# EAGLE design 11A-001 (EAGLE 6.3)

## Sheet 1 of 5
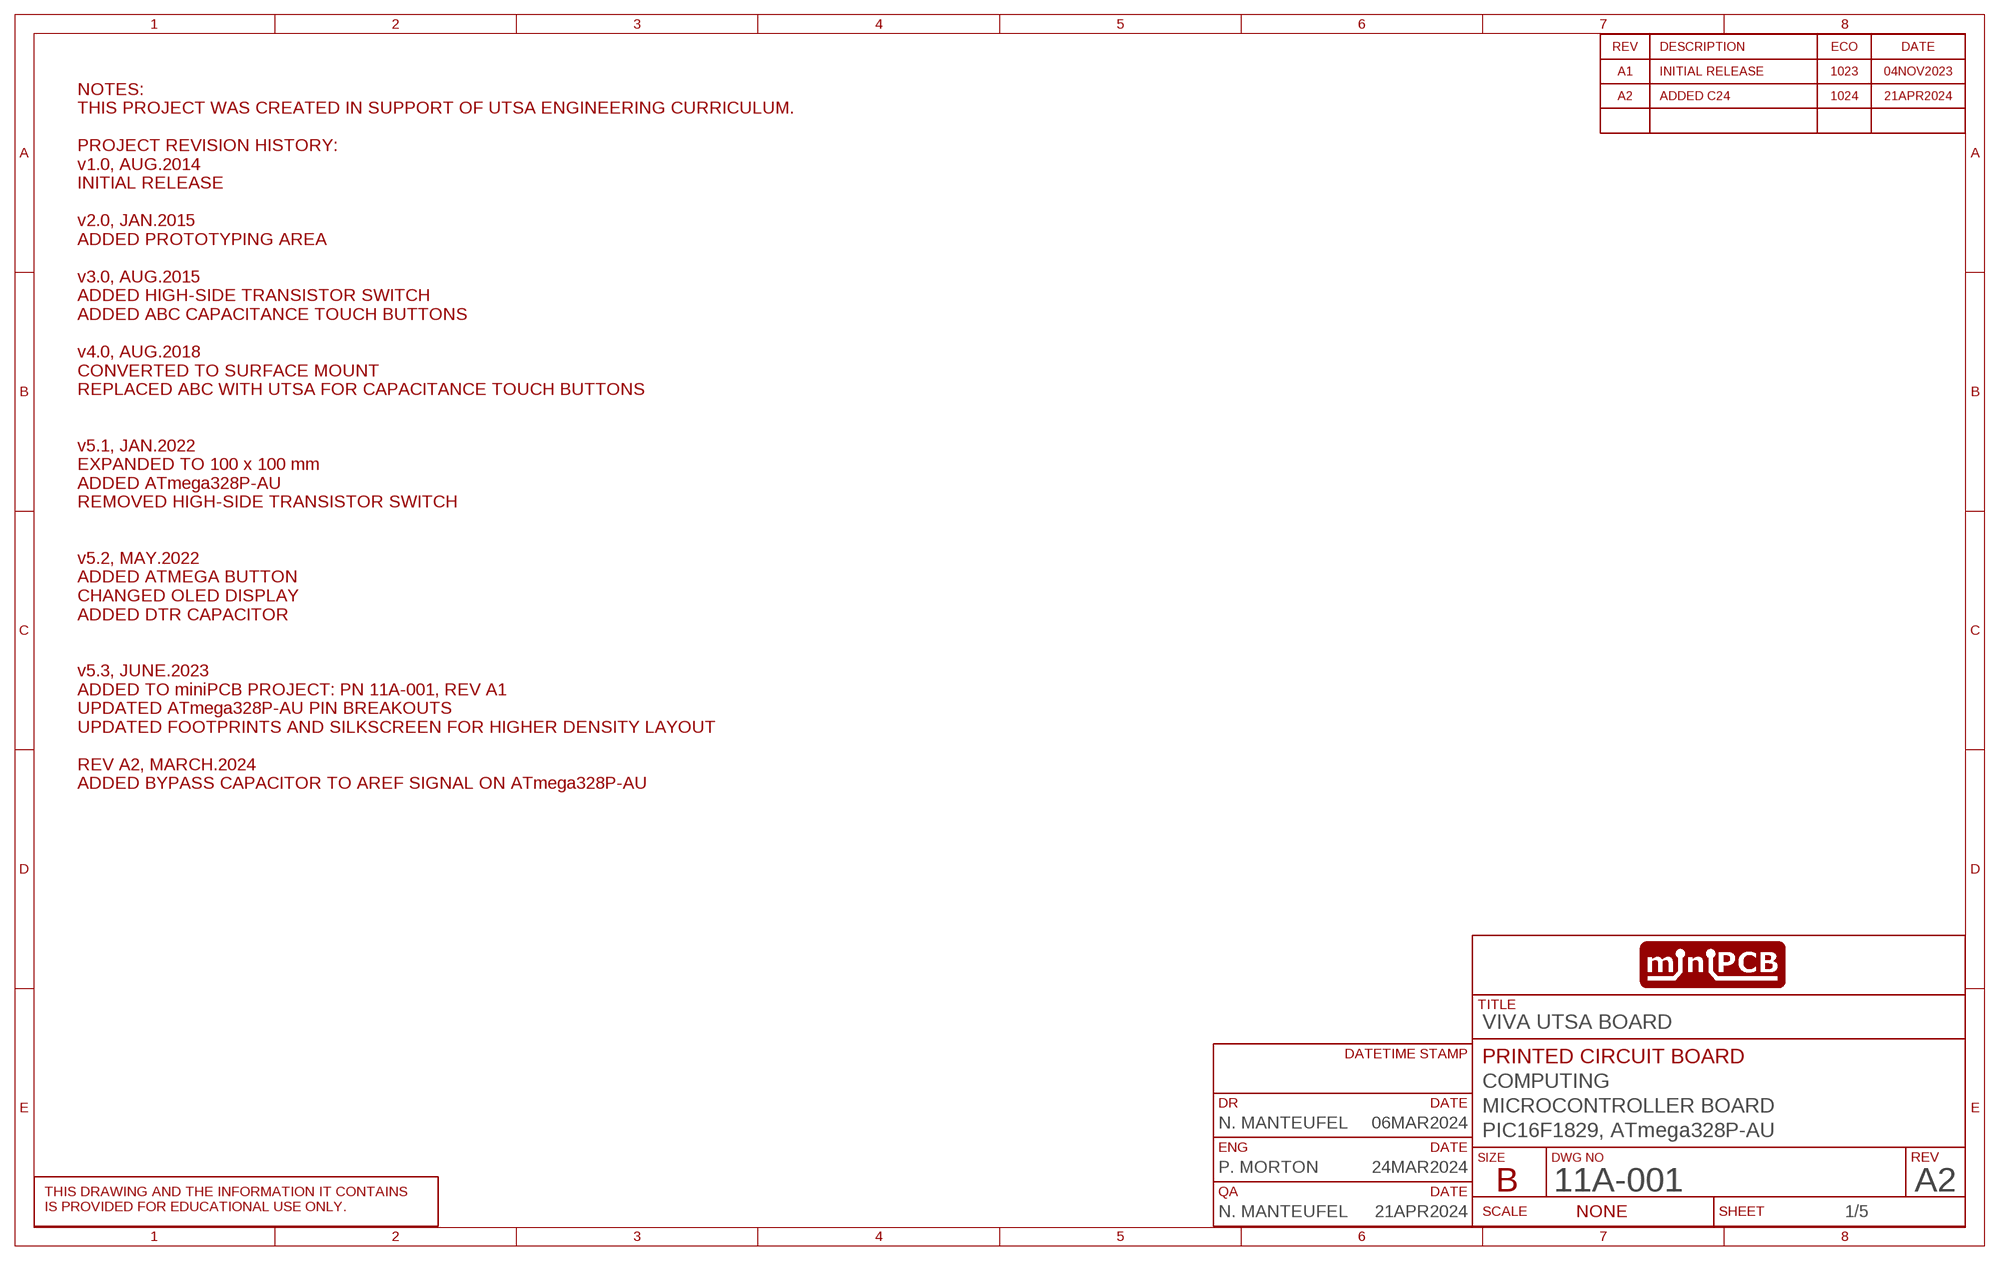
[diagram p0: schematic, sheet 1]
SHEET1 (SCHEMATIC): CIRCUIT_CATEGORY: COMPUTING; CIRCUIT_NAME: MICROCONTROLLER BOARD; CIRCUIT_VARIANT: PIC16F1829, ATmega328P-AU; DR: N. MANTEUFEL; DR_DATE: 06MAR2024; ENG: P. MORTON; ENG_DATE: 24MAR2024; PCB_PCBA: PRINTED CIRCUIT BOARD; QA: N. MANTEUFEL; QA_DATE: 21APR2024; REVA: A1; REVA_DATE: 04NOV2023; REVA_ECO: 1023; REVB: A2; REVB_DATE: 21APR2024; REVB_DESCRIPTION: ADDED C24; REVB_ECO: 1024; REVISION: A2; TITLE: VIVA UTSA BOARD

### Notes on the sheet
- NOTES:
  THIS PROJECT WAS CREATED IN SUPPORT OF UTSA ENGINEERING CURRICULUM.
  
  PROJECT REVISION HISTORY:
  v1.0, AUG.2014
  INITIAL RELEASE
  
  v2.0, JAN.2015
  ADDED PROTOTYPING AREA
  
  v3.0, AUG.2015
  ADDED HIGH-SIDE TRANSISTOR SWITCH
  ADDED ABC CAPACITANCE TOUCH BUTTONS
  
  v4.0, AUG.2018
  CONVERTED TO SURFACE MOUNT
  REPLACED ABC WITH UTSA FOR CAPACITANCE TOUCH BUTTONS
  
  
  v5.1, JAN.2022
  EXPANDED TO 100 x 100 mm
  ADDED ATmega328P-AU
  REMOVED HIGH-SIDE TRANSISTOR SWITCH
  
  
  v5.2, MAY.2022
  ADDED ATMEGA BUTTON
  CHANGED OLED DISPLAY
  ADDED DTR CAPACITOR
  
  
  v5.3, JUNE.2023
  ADDED TO miniPCB PROJECT: PN 11A-001, REV A1
  UPDATED ATmega328P-AU PIN BREAKOUTS
  UPDATED FOOTPRINTS AND SILKSCREEN FOR HIGHER DENSITY LAYOUT
  
  REV A2, MARCH.2024
  ADDED BYPASS CAPACITOR TO AREF SIGNAL ON ATmega328P-AU

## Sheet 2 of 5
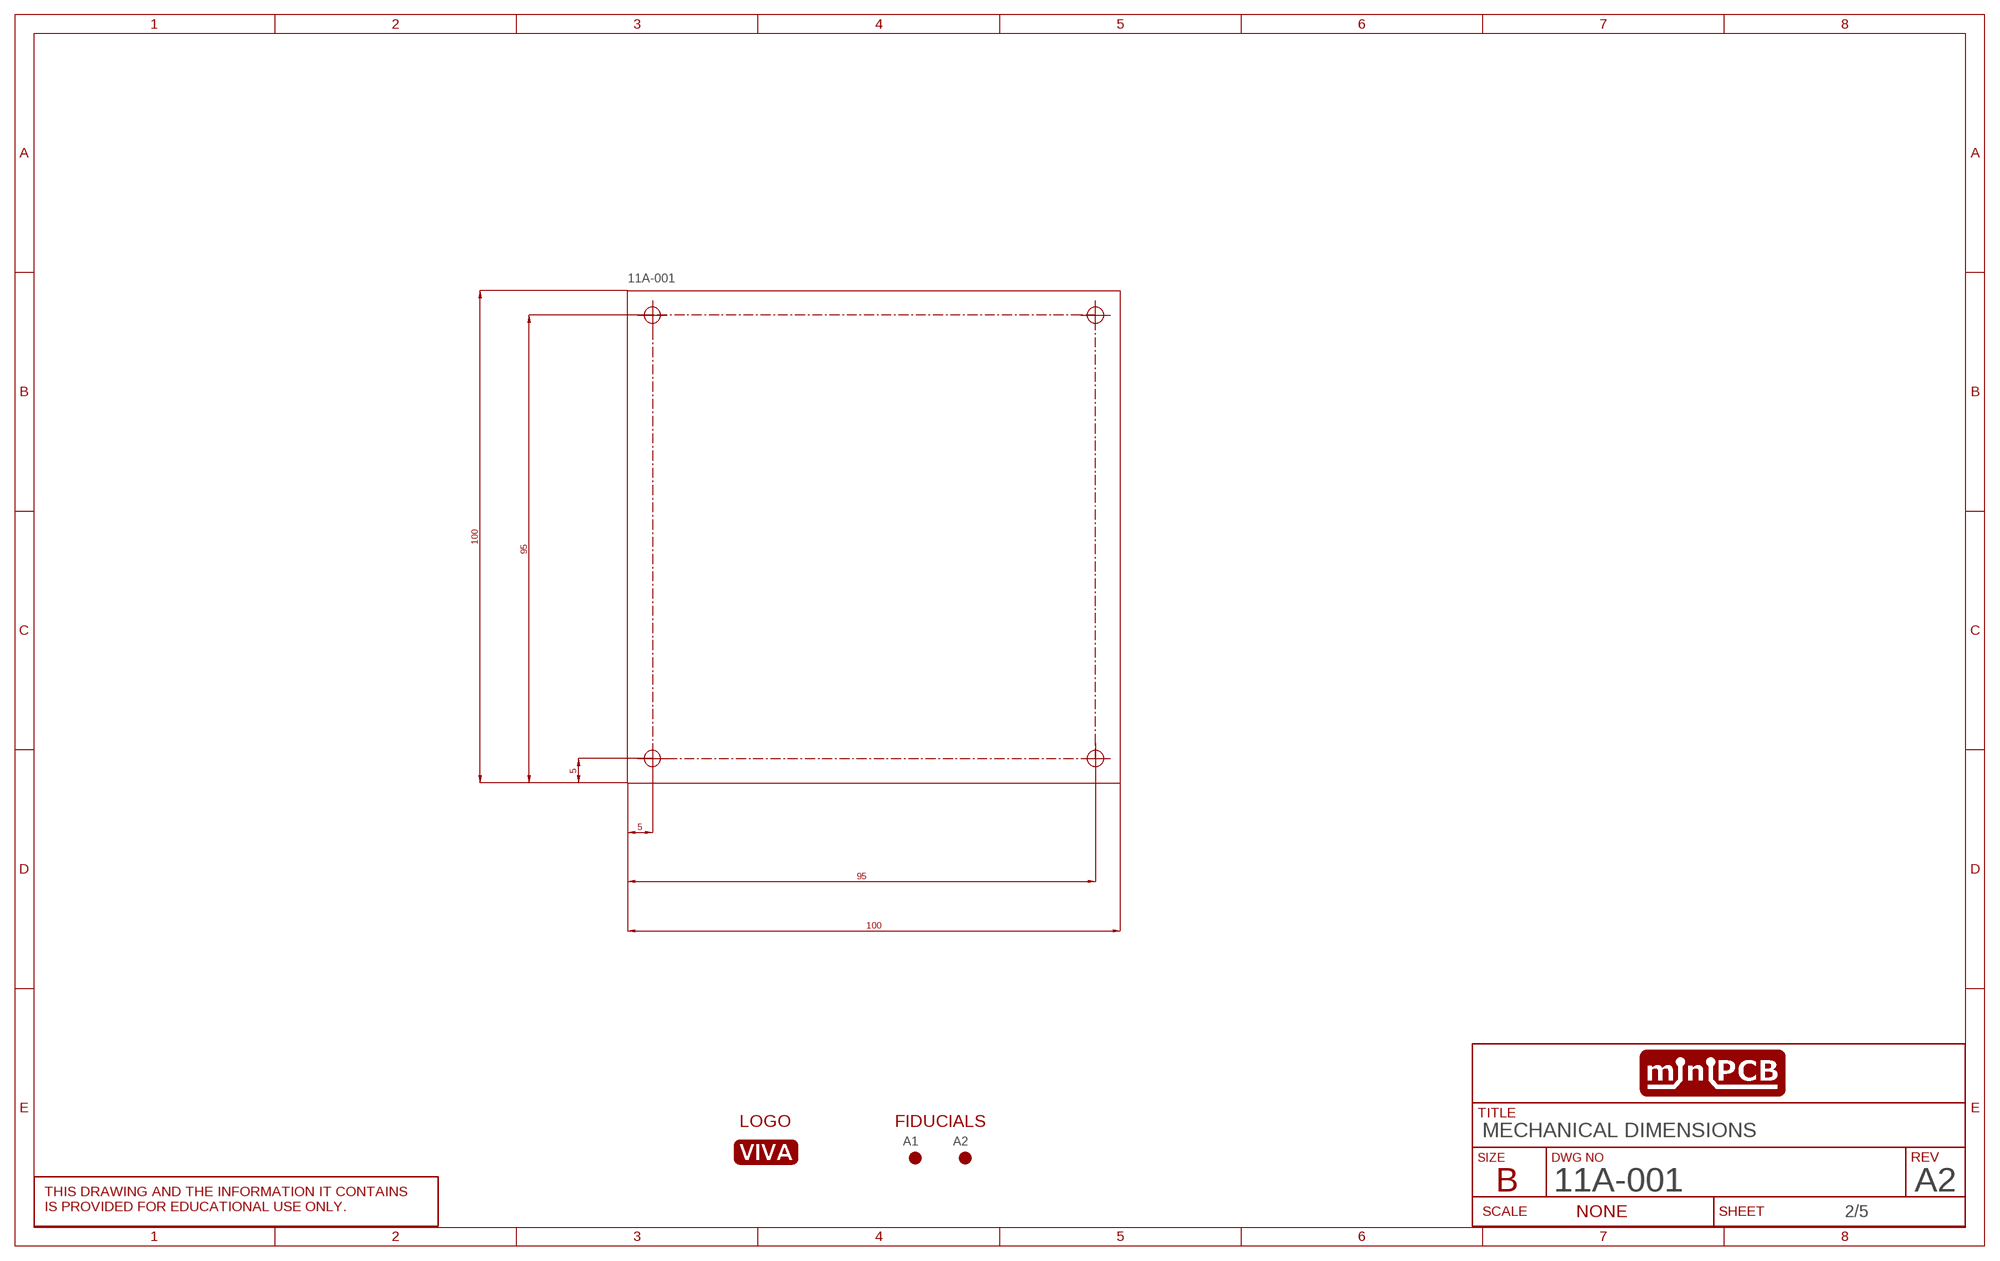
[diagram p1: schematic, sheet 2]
SHEET2 (SCHEMATIC): CIRCUIT_CATEGORY: COMPUTING; CIRCUIT_NAME: MICROCONTROLLER BOARD; CIRCUIT_VARIANT: PIC16F1829, ATmega328P-AU; DR: N. MANTEUFEL; DR_DATE: 31JUL2023; ENG: P. MORTON; ENG_DATE: 31JUL2023; PCB_PCBA: PRINTED CIRCUIT BOARD; REVA: A; REVISION: A2; TITLE: MECHANICAL DIMENSIONS

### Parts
-  11A-001  PCB_100X100  [PCB_100X100]
A1  FIDUCIAL  [FIDUCIAL]
A2  FIDUCIAL  [FIDUCIAL]
U$2  VIVA_LOGO  [VIVA_LOGO]

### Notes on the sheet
- LOGO | FIDUCIALS

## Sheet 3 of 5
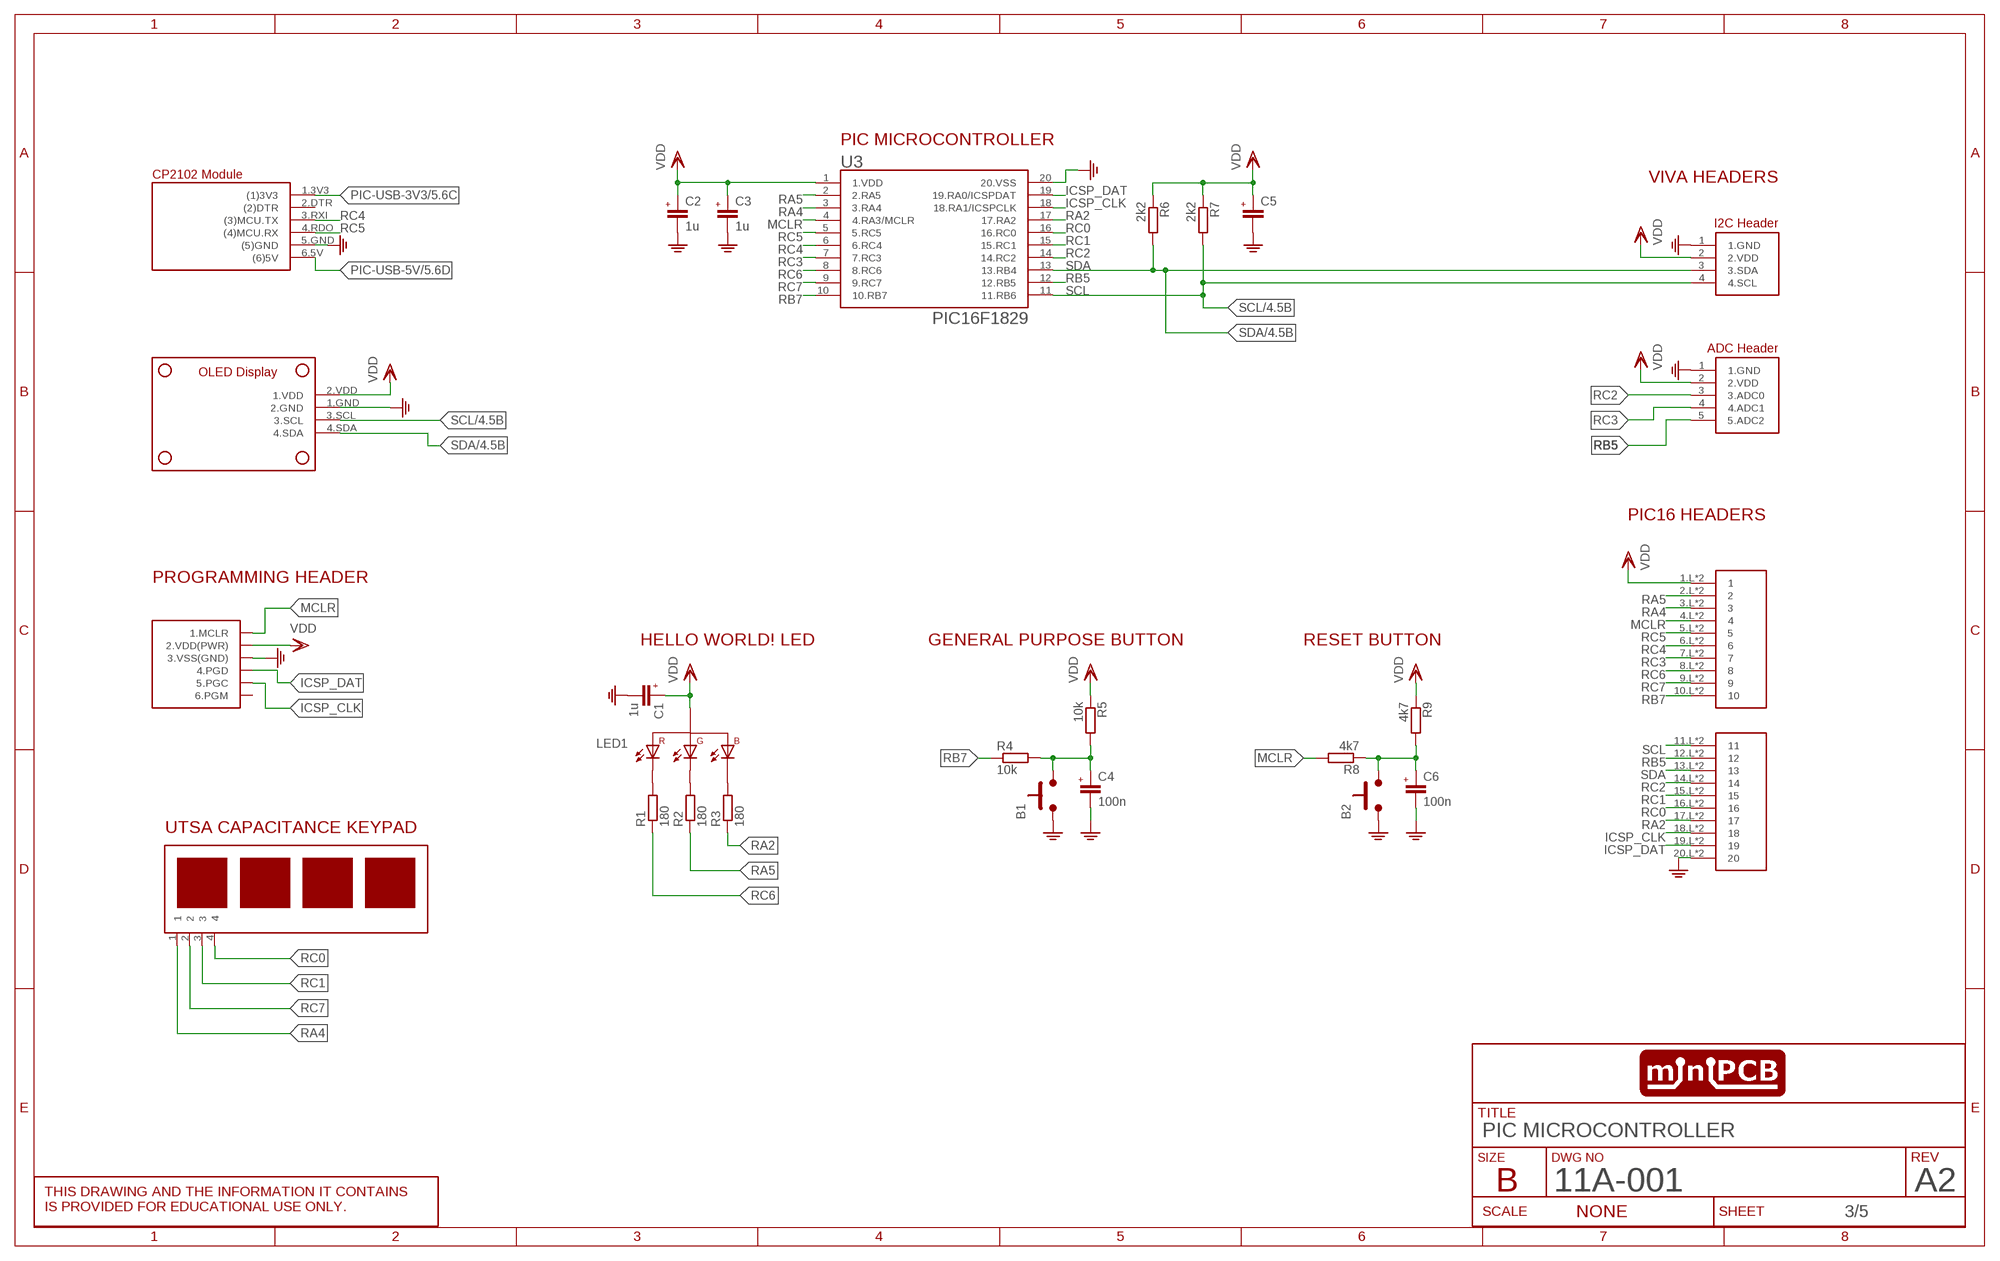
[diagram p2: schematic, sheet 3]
SHEET3 (SCHEMATIC): CIRCUIT_CATEGORY: COMPUTING; CIRCUIT_NAME: MICROCONTROLLER BOARD; CIRCUIT_VARIANT: PIC16F1829, ATmega328P-AU; DR: N. MANTEUFEL; DR_DATE: 31JUL2023; ENG: P. MORTON; ENG_DATE: 31JUL2023; PCB_PCBA: PRINTED CIRCUIT BOARD; REVA: A; REVISION: A2; TITLE: PIC MICROCONTROLLER

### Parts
$3_73_$  VIVA_OLEDGND  [VIVA_OLED-I2C-ALT]
B1  PUSHBUTTON6X6MM  [6X6MM]
B2  PUSHBUTTON6X6MM  [6X6MM]
C1  1u  C0805  [C0805]
C2  1u  C0805  [C0805]
C3  1u  C0805  [C0805]
C4  100n  C0805  [C0805]
C5  C0805  [C0805]
C6  100n  C0805  [C0805]
J1  PICKIT3  [PICKIT3]
J2  VIVA-HEADER-ADC-PIC16  [VIVA-HEADER-ADC-PIC16]
LED1  LED_RGBLTST-C19FD1WT  [0805_RGB]
R1  180  R-EU__R0805  [R0805]
R2  180  R-EU__R0805  [R0805]
R3  180  R-EU__R0805  [R0805]
R4  10k  R-EU__R0805  [R0805]
R5  10k  R-EU__R0805  [R0805]
R6  2k2  R-EU__R0805  [R0805]
R7  2k2  R-EU__R0805  [R0805]
R8  4k7  R-EU__R0805  [R0805]
R9  4k7  R-EU__R0805  [R0805]
U1  VIVA_UTSA-KEYPADV5  [VIVA_UTSA-KEYPAD-V5]
U2  VIVA_USB-TTL  [VIVA_USB_TTL_SUBTEXT]
U3  PIC16F1829  PIC16F1829300  [SOP20-NEW]
U4  VIVA-HEADER-I2C-RA  [VIVA-HEADER-I2C-RA]
U5  VIVA_PIC16BOARD  [VIVA_PIC16]

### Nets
B1-CAP: B1.3.B B1.4.B C4.1(+) R4.2 R5.2
GND: $3_73_$.1.GND(2.GND) B1.1.A B1.2.A B2.1.A B2.2.A C1.2(-) C2.2(-) C3.2(-) C4.2(-) C5.2(-) C6.2(-) J1.3(3.VSS(GND)) J2.1(1.GND) U2.5.GND((5)GND) U3.20(20.VSS) U4.1(1.GND) U5.20.L U5.20.R ; also sheet 4,5
ICSP_CLK: J1.5(5.PGC) U3.18(18.RA1/ICSPCLK) U5.18.L U5.18.R
ICSP_DAT: J1.4(4.PGD) U3.19(19.RA0/ICSPDAT) U5.19.L U5.19.R
MCLR: J1.1(1.MCLR) R8.2 U3.4(4.RA3/MCLR) U5.4.L U5.4.R
MCLR_CAP: B2.3.B B2.4.B C6.1(+) R8.1 R9.2
N$4: LED1.2(1.R-) R1.2
N$5: LED1.3(2.G-) R2.2
N$6: LED1.1(4.B-) R3.2
PIC-USB-3V3: U2.1.3V3((1)3V3) ; also sheet 5
PIC-USB-5V: U2.6.5V((6)5V) ; also sheet 5
RA2: R3.1 U3.17(17.RA2) U5.17.L U5.17.R
RA4: U1.1 U3.3(3.RA4) U5.3.L U5.3.R
RA5: R2.1 U3.2(2.RA5) U5.2.L U5.2.R
RB5: J2.5(5.ADC2) U3.12(12.RB5) U5.12.L U5.12.R
RB7: R4.1 U3.10(10.RB7) U5.10.L U5.10.R
RC0: U1.4 U3.16(16.RC0) U5.16.L U5.16.R
RC1: U1.3 U3.15(15.RC1) U5.15.L U5.15.R
RC2: J2.3(3.ADC0) U3.14(14.RC2) U5.14.L U5.14.R
RC3: J2.4(4.ADC1) U3.7(7.RC3) U5.7.L U5.7.R
RC4: U2.3.RXI((3)MCU.TX) U3.6(6.RC4) U5.6.L U5.6.R
RC5: U2.4.RDO((4)MCU.RX) U3.5(5.RC5) U5.5.L U5.5.R
RC6: R1.1 U3.8(8.RC6) U5.8.L U5.8.R
RC7: U1.2 U3.9(9.RC7) U5.9.L U5.9.R
SCL: $3_73_$.3.SCL R7.2 U3.11(11.RB6) U4.4(4.SCL) U5.11.L U5.11.R ; also sheet 4
SDA: $3_73_$.4.SDA R6.2 U3.13(13.RB4) U4.3(3.SDA) U5.13.L U5.13.R ; also sheet 4
VDD: $3_73_$.2.VDD(1.VDD) C1.1(+) C2.1(+) C3.1(+) C5.1(+) J1.2(2.VDD(PWR)) J2.2(2.VDD) LED1.4(3.+) R5.1 R6.1 R7.1 R9.1 U3.1(1.VDD) U4.2(2.VDD) U5.1.L U5.1.R ; also sheet 4,5
Unconnected: J1.6(6.PGM) U2.2.DTR((2)DTR)

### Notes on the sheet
- PIC MICROCONTROLLER
- VIVA HEADERS
- PIC16 HEADERS
- PROGRAMMING HEADER
- HELLO WORLD! LED | GENERAL PURPOSE BUTTON | RESET BUTTON
- UTSA CAPACITANCE KEYPAD

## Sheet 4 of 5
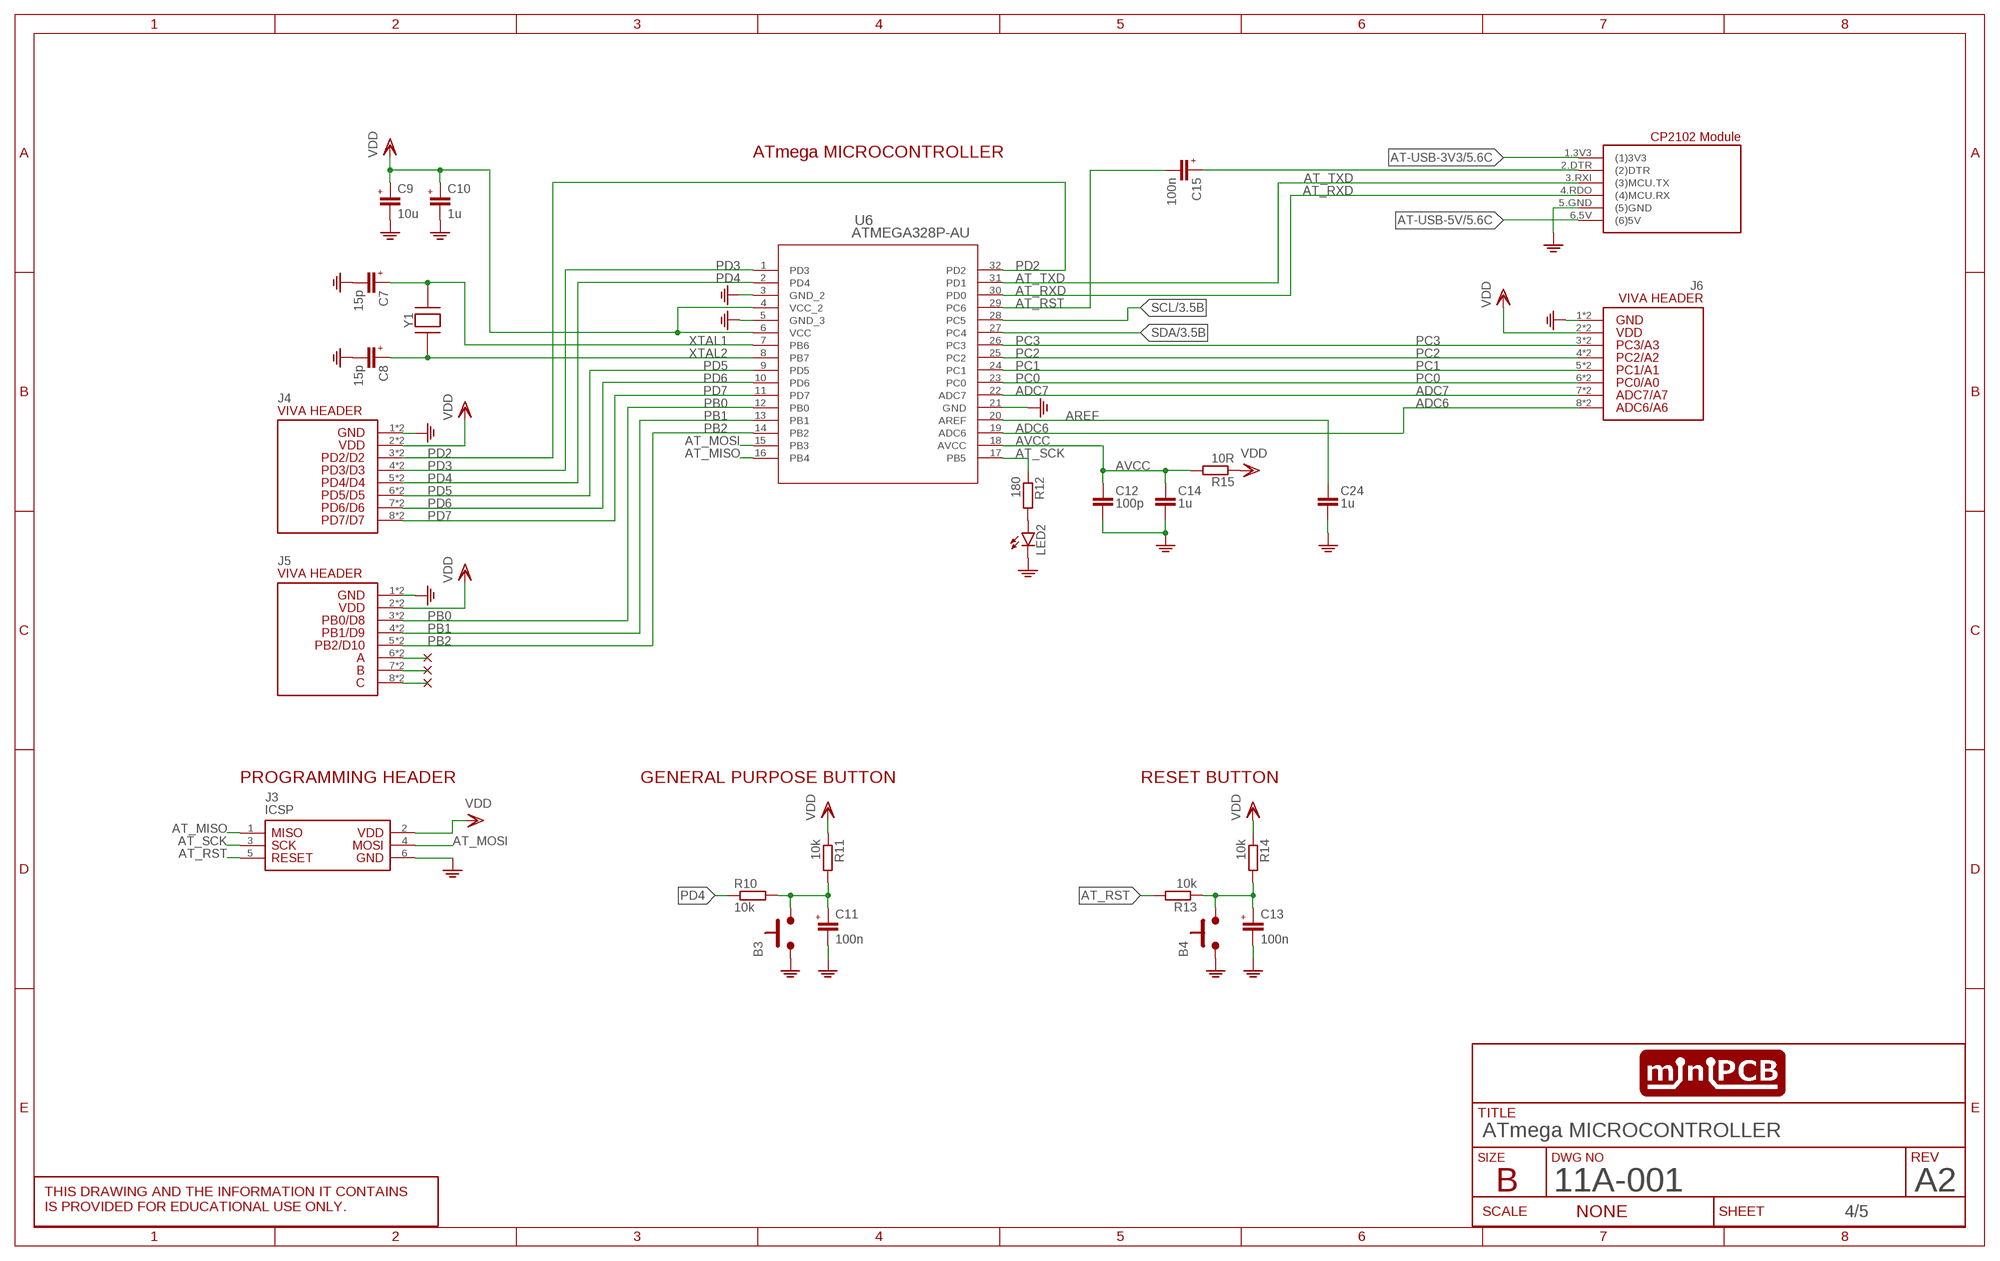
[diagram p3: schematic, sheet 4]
SHEET4 (SCHEMATIC): CIRCUIT_CATEGORY: COMPUTING; CIRCUIT_NAME: MICROCONTROLLER BOARD; CIRCUIT_VARIANT: PIC16F1829, ATmega328P-AU; DR: N. MANTEUFEL; DR_DATE: 31JUL2023; ENG: P. MORTON; ENG_DATE: 31JUL2023; PCB_PCBA: PRINTED CIRCUIT BOARD; REVA: A; REVISION: A2; TITLE: ATmega MICROCONTROLLER

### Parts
B3  PUSHBUTTON6X6MM  [6X6MM]
B4  PUSHBUTTON6X6MM  [6X6MM]
C7  15p  C0603  [C0603]
C8  15p  C0603  [C0603]
C9  10u  C0805  [C0805]
C10  1u  C0805  [C0805]
C11  100n  C0805  [C0805]
C12  100p  C-EU_C0805  [C0805]
C13  100n  C0805  [C0805]
C14  1u  C-EU_C0805  [C0805]
C15  100n  C0805  [C0805]
C24  1u  C-EU_C0805  [C0805]
J3  ICSP  PINS_6-2X3_AT  [PINS_6-2X3_AT]
J4  VIVA-HEADER-ADC-8P  [VIVA-HEADER-ADC-8P]
J5  VIVA-HEADER-ADC-8P  [VIVA-HEADER-ADC-8P]
J6  VIVA-HEADER-ADC-8P  [VIVA-HEADER-ADC-8P]
LED2  LEDSML0805  [SML0805]
R10  10k  R-EU__R0805  [R0805]
R11  10k  R-EU__R0805  [R0805]
R12  180  R-EU__R0805  [R0805]
R13  10k  R-EU__R0805  [R0805]
R14  10k  R-EU__R0805  [R0805]
R15  10R  R-EU__R0805  [R0805]
U6  ATMEGA328P-AU  ATMEGA328-AU  [32A_ATM]
U7  VIVA_USB-TTL  [VIVA_USB_TTL_SUBTEXT]
Y1  CRYSTAL-3225_4P  [TXC7M2]

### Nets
ADC6: J6.8(8.ADC5) J6.9(8.ADC5) U6.19(ADC6)
ADC7: J6.7(7.ADC4) J6.10(7.ADC4) U6.22(ADC7)
AREF: C24.1 U6.20(AREF)
AT-USB-3V3: U7.1.3V3((1)3V3) ; also sheet 5
AT-USB-5V: U7.6.5V((6)5V) ; also sheet 5
AT_DTR_CAP: C15.1(+) U7.2.DTR((2)DTR)
AT_MISO: J3.1 U6.16(PB4)
AT_MOSI: J3.4 U6.15(PB3)
AT_RST: C15.2(-) J3.5 R13.2 U6.29(PC6)
AT_RST_CAP: B4.3.B B4.4.B C13.1(+) R13.1 R14.2
AT_RXD: U6.30(PD0) U7.4.RDO((4)MCU.RX)
AT_SCK: J3.3 R12.1 U6.17(PB5)
AT_TXD: U6.31(PD1) U7.3.RXI((3)MCU.TX)
AVCC: C12.1 C14.1 R15.2 U6.18(AVCC)
GND: B3.1.A B3.2.A B4.1.A B4.2.A C7.1(-) C8.1(-) C9.2(-) C10.2(-) C11.2(-) C12.2 C13.2(-) C14.2 C24.2 J3.6 J4.1(1.GND) J4.16(1.GND) J5.1(1.GND) J5.16(1.GND) J6.1(1.GND) J6.16(1.GND) LED2.C U6.3(GND_2) U6.5(GND_3) U6.21(GND) U7.5.GND((5)GND) ; also sheet 3,5
N$33: J5.6(6.ADC3) J5.11(6.ADC3)
N$34: J5.7(7.ADC4) J5.10(7.ADC4)
N$35: J5.8(8.ADC5) J5.9(8.ADC5)
N$37: LED2.A R12.2
PB0: J5.3(3.ADC0) J5.14(3.ADC0) U6.12(PB0)
PB1: J5.4(4.ADC1) J5.13(4.ADC1) U6.13(PB1)
PB2: J5.5(5.ADC2) J5.12(5.ADC2) U6.14(PB2)
PC0: J6.6(6.ADC3) J6.11(6.ADC3) U6.23(PC0)
PC1: J6.5(5.ADC2) J6.12(5.ADC2) U6.24(PC1)
PC2: J6.4(4.ADC1) J6.13(4.ADC1) U6.25(PC2)
PC3: J6.3(3.ADC0) J6.14(3.ADC0) U6.26(PC3)
PD2: J4.3(3.ADC0) J4.14(3.ADC0) U6.32(PD2)
PD3: J4.4(4.ADC1) J4.13(4.ADC1) U6.1(PD3)
PD4: J4.5(5.ADC2) J4.12(5.ADC2) R10.1 U6.2(PD4)
PD4-CAP: B3.3.B B3.4.B C11.1(+) R10.2 R11.2
PD5: J4.6(6.ADC3) J4.11(6.ADC3) U6.9(PD5)
PD6: J4.7(7.ADC4) J4.10(7.ADC4) U6.10(PD6)
PD7: J4.8(8.ADC5) J4.9(8.ADC5) U6.11(PD7)
SCL: U6.28(PC5) ; also sheet 3
SDA: U6.27(PC4) ; also sheet 3
VDD: C9.1(+) C10.1(+) J3.2 J4.2(2.VDD) J4.15(2.VDD) J5.2(2.VDD) J5.15(2.VDD) J6.2(2.VDD) J6.15(2.VDD) R11.1 R14.1 R15.1 U6.4(VCC_2) U6.6(VCC) ; also sheet 3,5
XTAL1: C7.2(+) U6.7(PB6) Y1.3
XTAL2: C8.2(+) U6.8(PB7) Y1.1

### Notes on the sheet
- ATmega MICROCONTROLLER
- PROGRAMMING HEADER | GENERAL PURPOSE BUTTON | RESET BUTTON

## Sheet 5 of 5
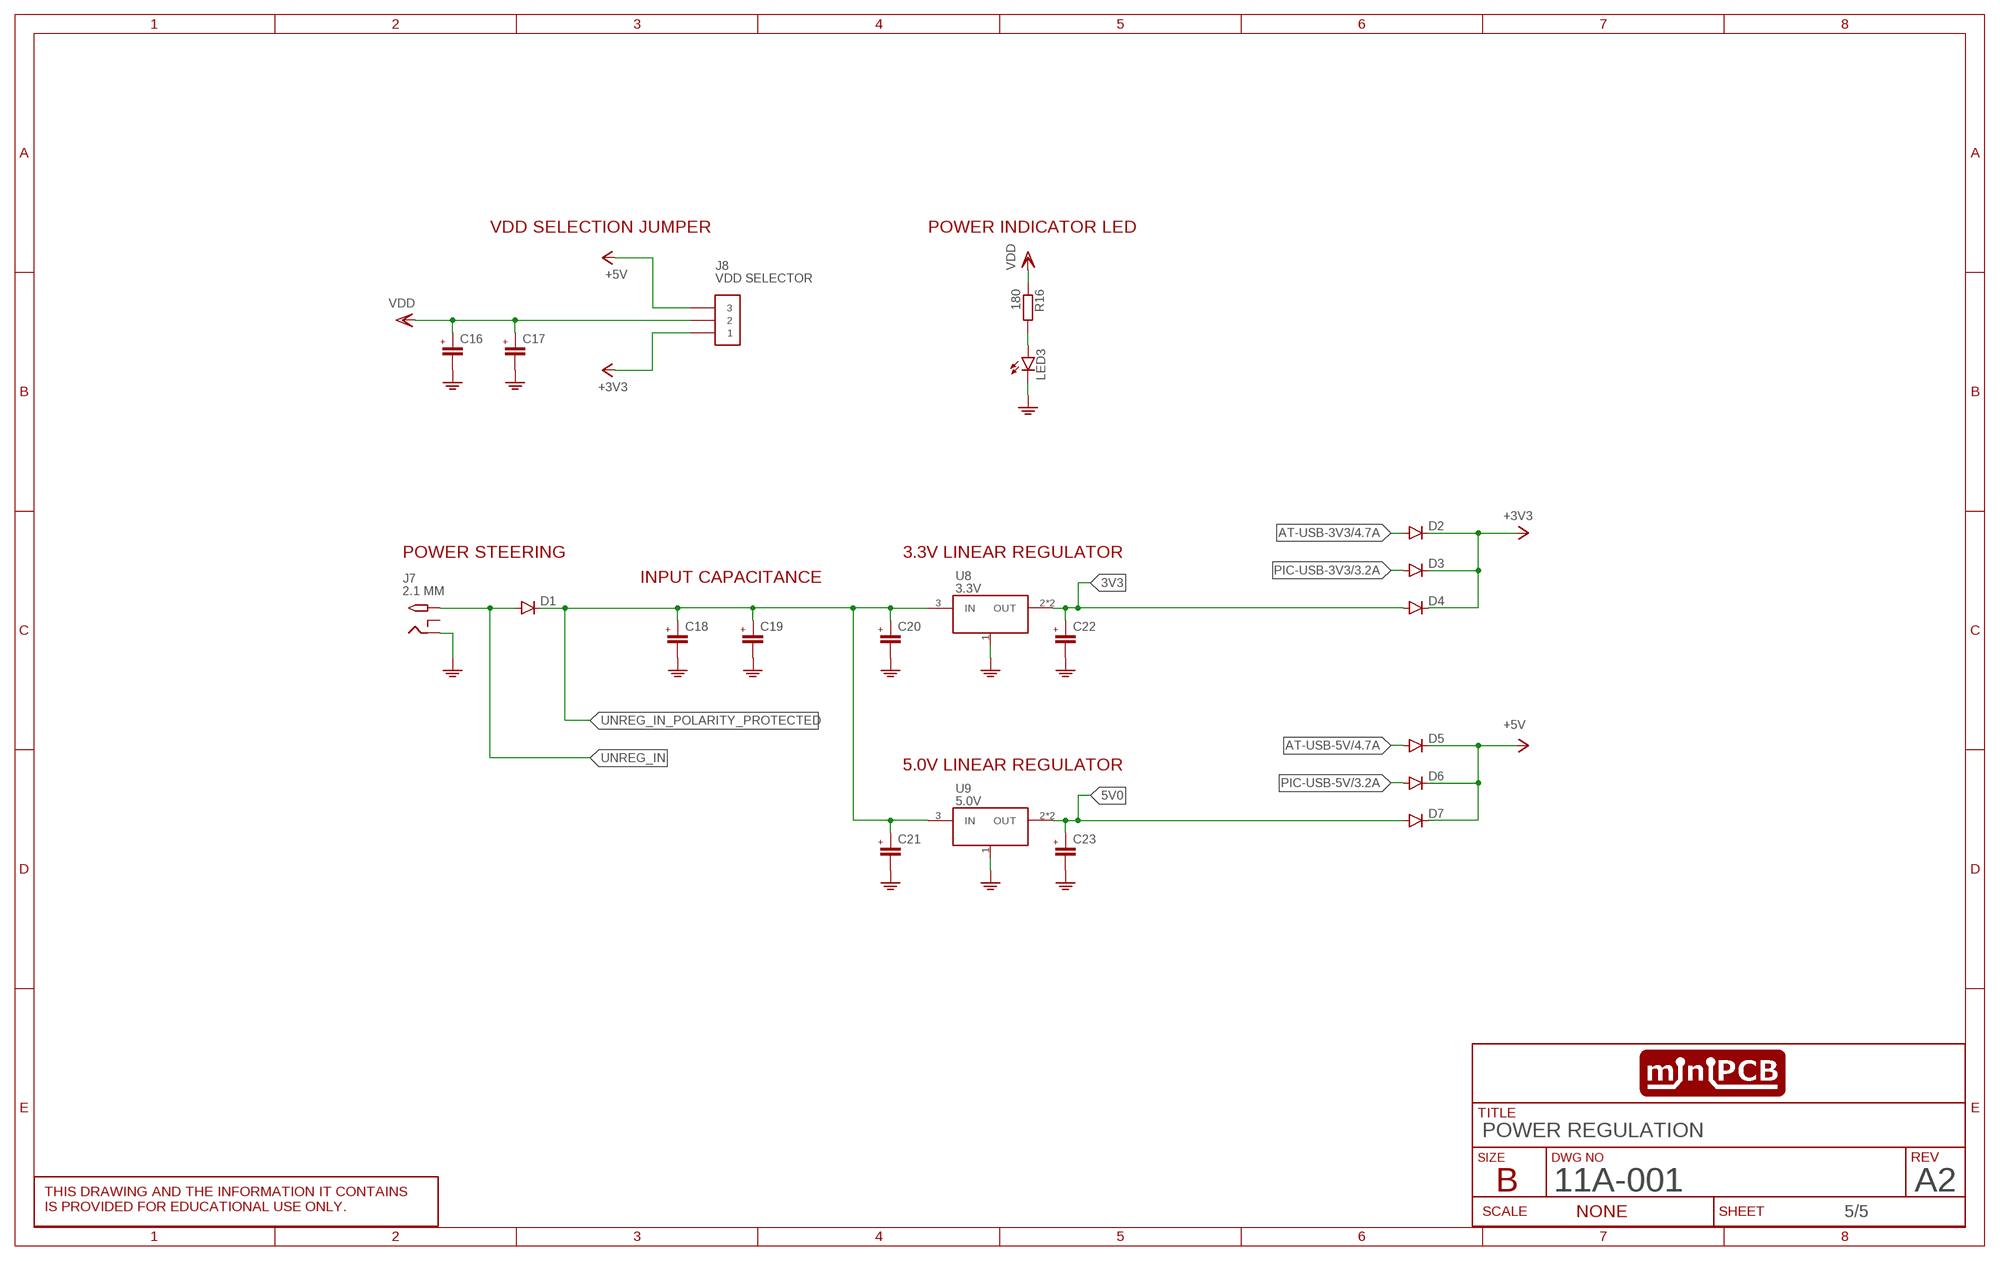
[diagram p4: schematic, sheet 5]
SHEET5 (SCHEMATIC): CIRCUIT_CATEGORY: COMPUTING; CIRCUIT_NAME: MICROCONTROLLER BOARD; CIRCUIT_VARIANT: PIC16F1829, ATmega328P-AU; DR: N. MANTEUFEL; DR_DATE: 31JUL2023; ENG: P. MORTON; ENG_DATE: 31JUL2023; PCB_PCBA: PRINTED CIRCUIT BOARD; REVA: A; REVISION: A2; TITLE: POWER REGULATION

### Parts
C16  C0805  [C0805]
C17  C0805  [C0805]
C18  C0805  [C0805]
C19  C0805  [C0805]
C20  C0805  [C0805]
C21  C0805  [C0805]
C22  C0805  [C0805]
C23  C0805  [C0805]
D1  DIODE-DO214AC  [DO214AC]
D2  DIODE-DO214AC  [DO214AC]
D3  DIODE-DO214AC  [DO214AC]
D4  DIODE-DO214AC  [DO214AC]
D5  DIODE-DO214AC  [DO214AC]
D6  DIODE-DO214AC  [DO214AC]
D7  DIODE-DO214AC  [DO214AC]
J7  2.1 MM  2.1MMJACKTHM  [PJ-102A]
J8  VDD SELECTOR  PINS_3_2.54  [PINS_3]
LED3  LEDSML0805  [SML0805]
R16  180  R-EU__R0805  [R0805]
U8  3.3V  REGULATOR_SCHLM1117  [SOT223]
U9  5.0V  REGULATOR_SCHLM1117  [SOT223]

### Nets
3V3: C22.1(+) D4.A U8.2(OUT) U8.4.TAB(OUT)
5V0: C23.1(+) D7.A U9.2(OUT) U9.4.TAB(OUT)
+3V3: D2.C D3.C D4.C J8.1
+5V: D5.C D6.C D7.C J8.3
AT-USB-3V3: D2.A ; also sheet 4
AT-USB-5V: D5.A ; also sheet 4
GND: C16.2(-) C17.2(-) C18.2(-) C19.2(-) C20.2(-) C21.2(-) C22.2(-) C23.2(-) J7.RING LED3.C U8.1(GND) U9.1(GND) ; also sheet 3,4
LED_POWER: LED3.A R16.2
PIC-USB-3V3: D3.A ; also sheet 3
PIC-USB-5V: D6.A ; also sheet 3
UNREG_IN: D1.A J7.TIP
UNREG_IN_POLARITY_PROTECTED: C18.1(+) C19.1(+) C20.1(+) C21.1(+) D1.C U8.3(IN) U9.3(IN)
VDD: C16.1(+) C17.1(+) J8.2 R16.1 ; also sheet 3,4
Unconnected: J7.RING_SW

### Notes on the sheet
- VDD SELECTION JUMPER | POWER INDICATOR LED
- POWER STEERING | 3.3V LINEAR REGULATOR
- INPUT CAPACITANCE
- 5.0V LINEAR REGULATOR

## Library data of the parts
$3_73_$ = utsa:VIVA_OLED
- = utsa:PCB_100X100
A1 A2 = utsa:FIDUCIAL
B1-B4 = nolan-utsa:PUSHBUTTON: Tactile push button switch
C1-C11 C13 C15-C23 = utsa:C
C12 C14 C24 = utsa:C-EU: CAPACITOR, European symbol
D1-D7 = utsa:DIODE-: DIODE
J1 = nolan-viva:PICKIT3
J2 = utsa:VIVA-HEADER-ADC
J3 = utsa:PINS_6-2X3_AT; P1: MISO; P2: VDD; P3: SCK; P4: MOSI; P5: RESET; P6: GND
J4 = utsa:VIVA-HEADER-ADC-8P; P3: PD2/D2; P4: PD3/D3; P5: PD4/D4; P6: PD5/D5; P7: PD6/D6; P8: PD7/D7
J5 = utsa:VIVA-HEADER-ADC-8P; P3: PB0/D8; P4: PB1/D9; P5: PB2/D10; P6: A; P7: B; P8: C
J6 = utsa:VIVA-HEADER-ADC-8P; P3: PC3/A3; P4: PC2/A2; P5: PC1/A1; P6: PC0/A0; P7: ADC7/A7; P8: ADC6/A6
J7 = utsa:2.1MMJACK: 2.1mm x 5.5mm THM DC jack with internal switch. Digikey part #PJ-102A, 4UCON part #05537 2.1mm x 5.5mm SMT DC jack with internal switch. Digikey part #PJ-002A-SMT, 4UCON part #03267 By microbuilder.eu & adafruit.com
J8 = utsa:PINS_3
LED1 = utsa:LED_RGB
LED2 LED3 = utsa:LED: LED
R1-R16 = utsa:R-EU_: RESISTOR, European symbol
U1 = utsa:VIVA_UTSA-KEYPAD
U2 U7 = utsa:VIVA_USB-TTL
U3 = utsa:PIC16F1829
U4 = utsa:VIVA-HEADER-I2C
U5 = utsa:VIVA_PIC16
U6 = utsa:ATMEGA328-AU; COPYRIGHT: Copyright (C) 2021 Ultra Librarian. All rights reserved.; MANUFACTURER_PART_NUMBER: ATMEGA328-AU; MFR_NAME: Microchip
U8 U9 = utsa:REGULATOR_SCH: Linear Regulator in SOT-223 package. NOTE: select correct pinout for your application. Tab may be OUT or GND!
U$2 = utsa:VIVA_LOGO
Y1 = utsa:CRYSTAL: HC49S Crystal Oscillator

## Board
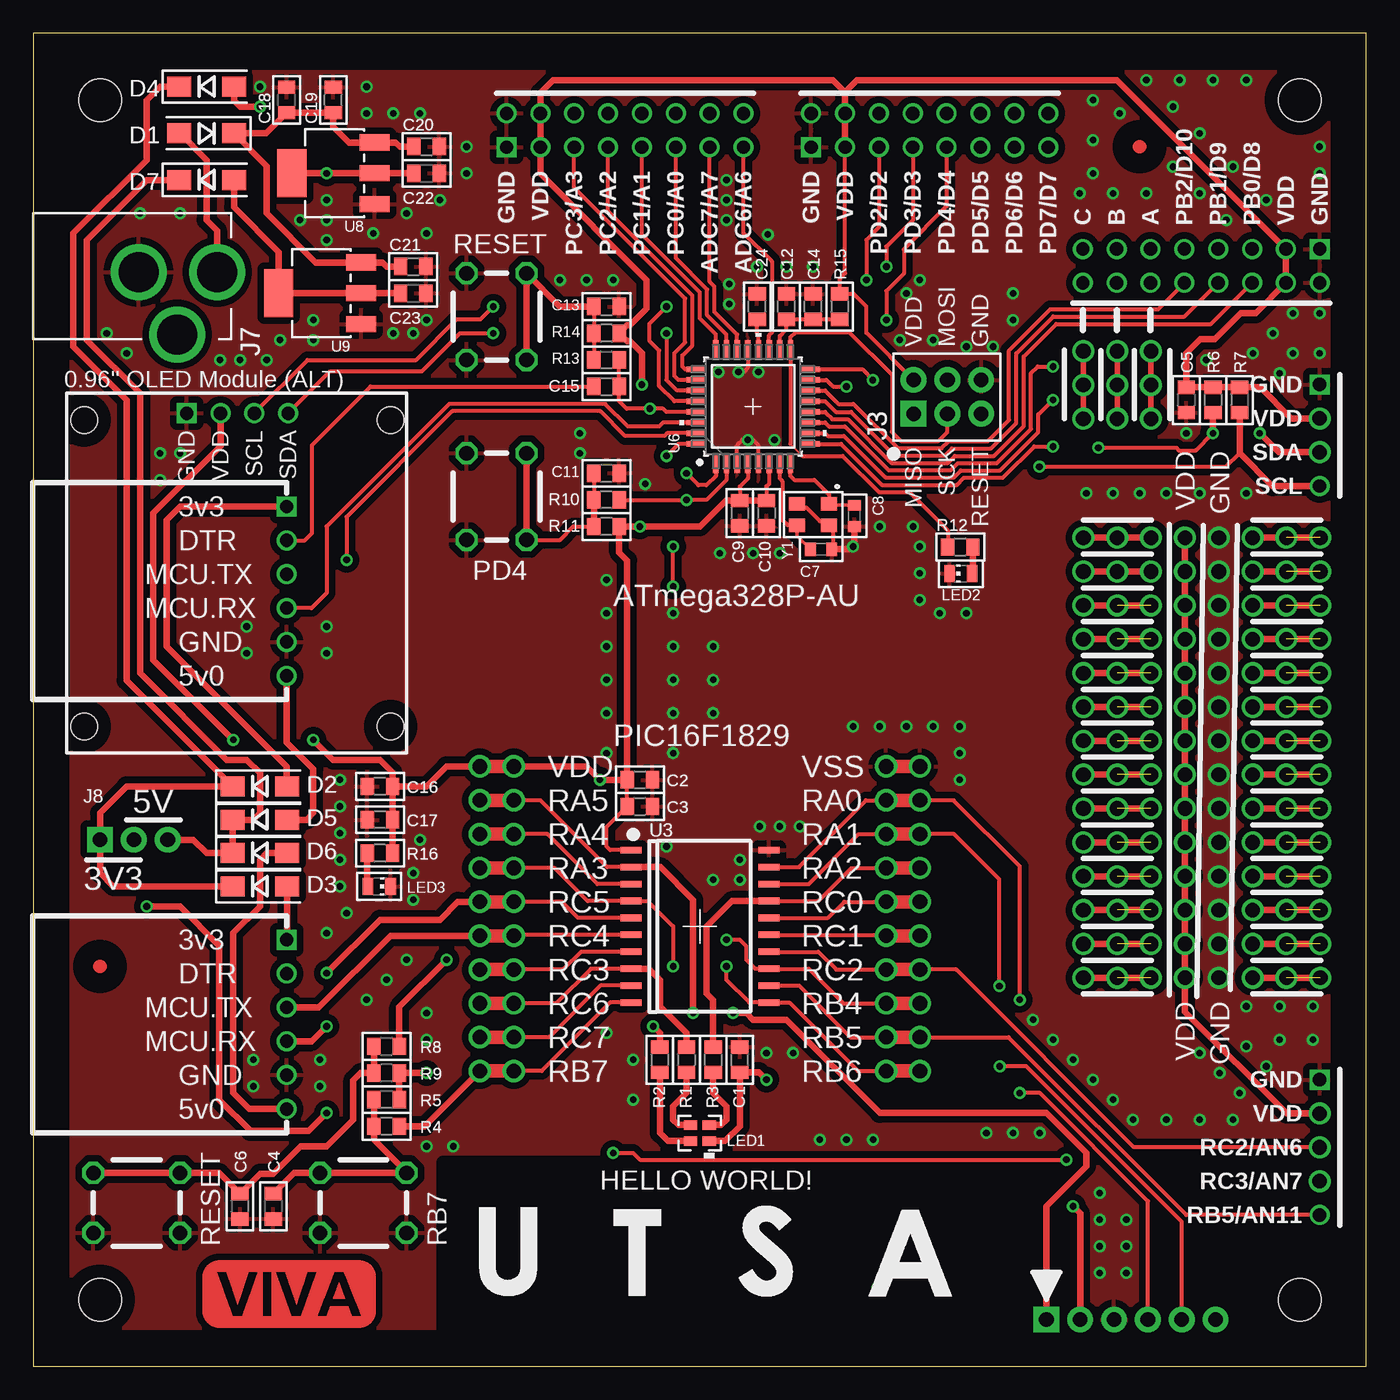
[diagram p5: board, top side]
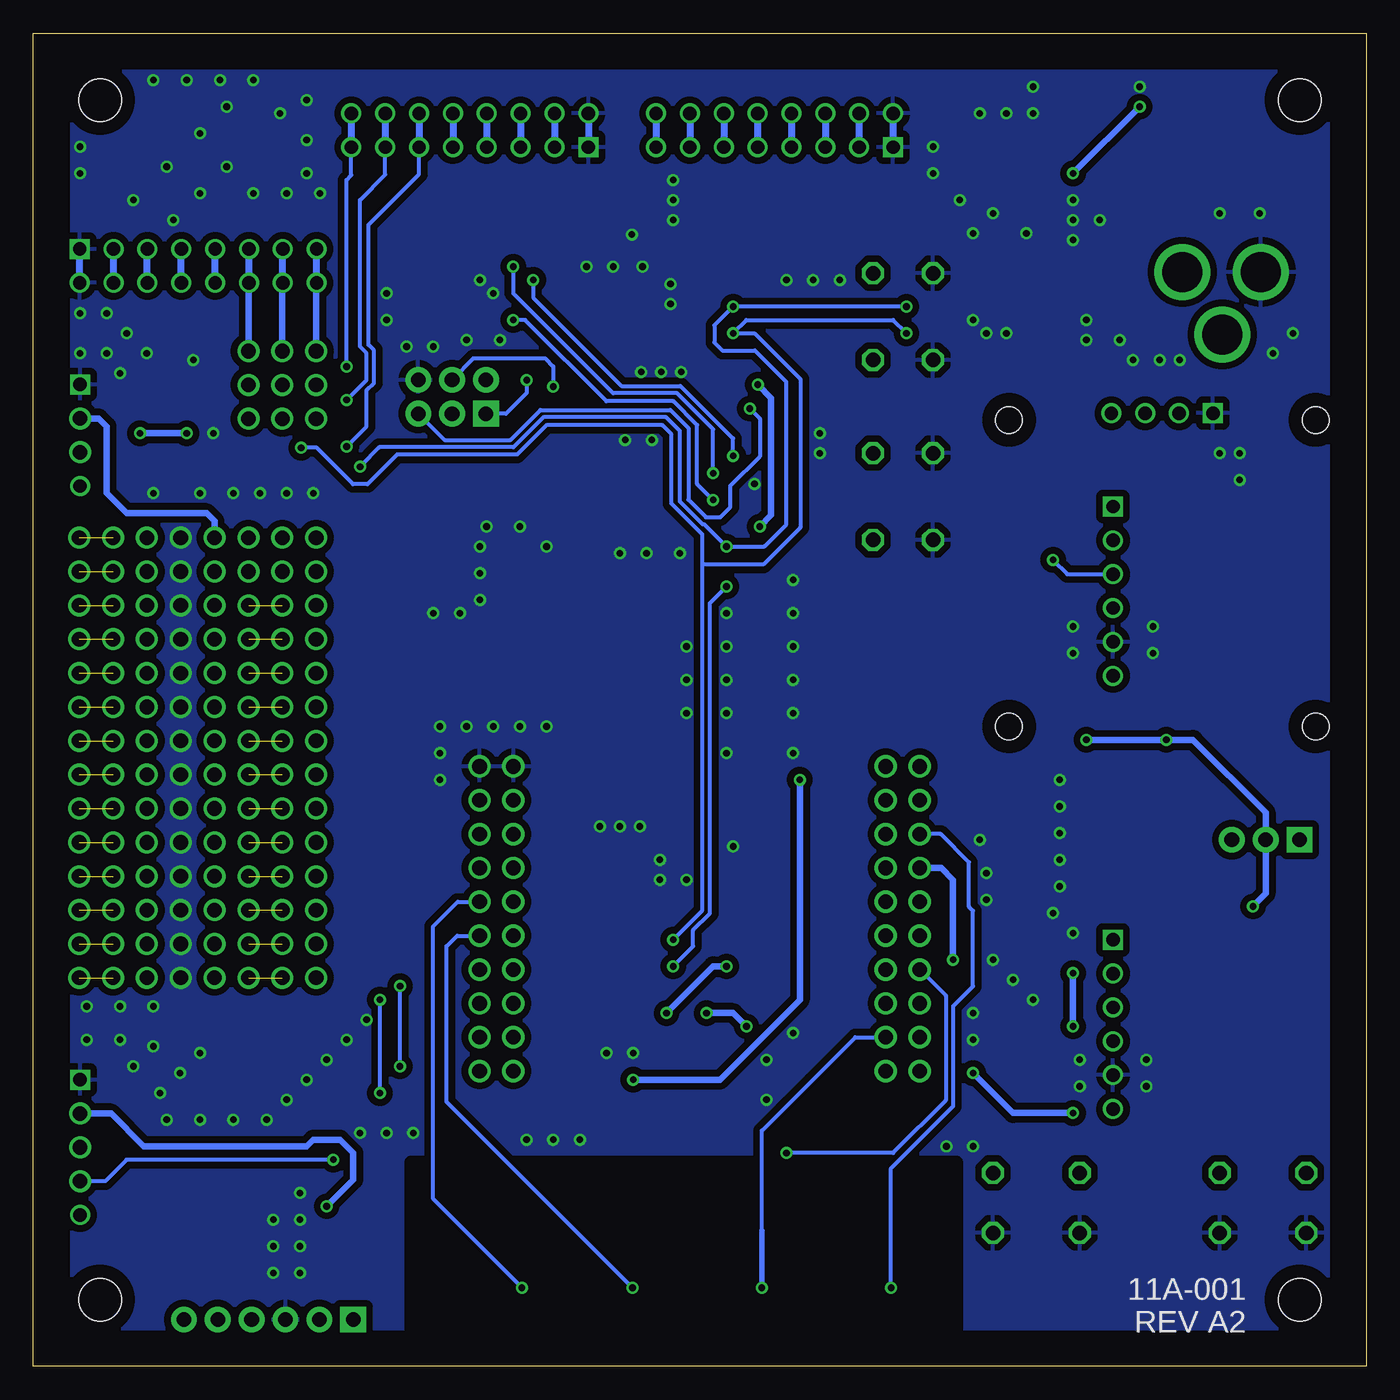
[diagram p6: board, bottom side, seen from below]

Size 100 x 100 mm. Coordinates in mm from the lower left corner, seen from the top.
Copper layers (1*16): Top 0.035mm / dielectric 1.5mm / Bottom 0.035mm
Design rules "minipcb": minimum track width 0.2mm, minimum drill 0.5mm, track to track 0.25mm, track to pad 0.5mm, pad to pad 0.5mm, via to via 0.5mm, smd to smd 0.15mm, copper to edge 1mm, drill to drill 1mm, minimum pad ring 0.2mm, minimum via ring 0.2mm, stop-mask expansion 0.1mm, vias tented up to drill 0.6mm, thermal gap 0.5mm

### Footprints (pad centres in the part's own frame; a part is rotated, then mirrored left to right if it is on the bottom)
VIVA_OLED-I2C-ALT = drill 1 square: 1.GND 0,0 | drill 1: 2.VDD 2.54,0; 3.SCL 5.08,0; 4.SDA 7.62,0 | hole 2: -7.7,-0.5; 15.3,-0.5; -7.7,-23.5; 15.3,-23.5
PCB_100X100 = hole 3.2: 5,95; 95,95; 95,5; 5,5
FIDUCIAL = smd 0 x 0: FIDUCIAL 0,0
6X6MM = drill 1.1 octagon: 1.A 0,0; 2.A 6.5,0; 3.B 0,4.5; 4.B 6.5,4.5
C0805 = smd 1 x 1.3: 1 -0.95,0; 2 0.95,0
C0603 = smd 0.8 x 1: 1 -0.8,0; 2 0.8,0
DO214AC = smd 1.8 x 1.5: A 2.05,0; C -2.05,0
PICKIT3 = drill 1.1 pad 1.93 square: 1 0,0 | drill 1.1 pad 1.93: 2 2.54,0; 3 5.08,0; 4 7.62,0; 5 10.16,0; 6 12.7,0
VIVA-HEADER-ADC-PIC16 = drill 1 square: 1 0,0 | drill 1.1: 2 2.54,0; 3 5.08,0; 4 7.62,0 | drill 1: 5 10.16,0
PINS_6-2X3_AT = drill 1.1 pad 1.93 square: 1 0,0 | drill 1.1 pad 1.93: 2 2.54,0; 3 0,-2.54; 4 2.54,-2.54; 5 0,-5.08; 6 2.54,-5.08
VIVA-HEADER-ADC-8P = drill 1 square: 1 0,0 | drill 1: 2 2.54,0; 3 5.08,0; 4 7.62,0; 5 10.16,0; 6 12.7,0; 7 15.24,0; 8 17.78,0; 9 17.78,2.54; 10 15.24,2.54; 11 12.7,2.54; 12 10.16,2.54; 13 7.62,2.54; 14 5.08,2.54; 15 2.54,2.54; 16 0,2.54
PJ-102A = drill 3 pad 4: RING 0.1,-3.39; RING_SW -4.6,-6.29; TIP 0.1,-9.29
PINS_3 = drill 1.1 pad 1.93 square: 1 0,0 | drill 1.1 pad 1.93: 2 2.54,0; 3 5.08,0
0805_RGB = smd 1 x 0.7: 1 0.7,0.6; 2 -0.7,0.6; 3 -0.7,-0.6; 4 0.7,-0.6
SML0805 = smd 0.8 x 1.27: A -0.9,0; C 0.8,0
R0805 = smd 1 x 1.3: 1 -0.95,0; 2 0.95,0
VIVA_UTSA-KEYPAD-V5 = drill 0.5: 1 -14.36,4.38; 2 -4.66,4.38; 3 5.04,4.38; 4 13.34,4.38
VIVA_USB_TTL_SUBTEXT = drill 1 square: 1.3V3 0,0 | drill 1: 2.DTR 0,-2.54; 3.RXI 0,-5.08; 4.RDO 0,-7.62; 5.GND 0,-10.16; 6.5V 0,-12.7
SOP20-NEW = smd 0.5 x 1.6: 1 -5.715,-5.152; 2 -4.445,-5.152; 3 -3.175,-5.152; 4 -1.905,-5.152; 5 -0.635,-5.152; 6 0.635,-5.152; 7 1.905,-5.152; 8 3.175,-5.152; 9 4.445,-5.152; 10 5.715,-5.152; 11 5.715,5.188; 12 4.445,5.188; 13 3.175,5.188; 14 1.905,5.188; 15 0.635,5.188; 16 -0.635,5.188; 17 -1.905,5.188; 18 -3.175,5.188; 19 -4.445,5.188; 20 -5.715,5.188
VIVA-HEADER-I2C-RA = drill 1 square: 1 0,0 | drill 1.1: 2 2.54,0; 3 5.08,0 | drill 1: 4 7.62,0
VIVA_PIC16 = drill 1.1 pad 1.676: 1.L 0,0; 1.R 2.54,0; 2.L 0,-2.54; 2.R 2.54,-2.54; 3.L 0,-5.08; 3.R 2.54,-5.08; 4.L 0,-7.62; 4.R 2.54,-7.62; 5.L 0,-10.16; 5.R 2.54,-10.16; 6.L 0,-12.7; 6.R 2.54,-12.7; 7.L 0,-15.24; 7.R 2.54,-15.24; 8.L 0,-17.78; 8.R 2.54,-17.78; 9.L 0,-20.32; 9.R 2.54,-20.32; 10.L 0,-22.86; 10.R 2.54,-22.86; 11.L 30.48,-22.86; 11.R 33.02,-22.86; 12.L 30.48,-20.32; 12.R 33.02,-20.32; 13.L 30.48,-17.78; 13.R 33.02,-17.78; 14.L 30.48,-15.24; 14.R 33.02,-15.24; 15.L 30.48,-12.7; 15.R 33.02,-12.7; 16.L 30.48,-10.16; 16.R 33.02,-10.16; 17.L 30.48,-7.62; 17.R 33.02,-7.62; 18.L 30.48,-5.08; 18.R 33.02,-5.08; 19.L 30.48,-2.54; 19.R 33.02,-2.54; 20.L 30.48,0; 20.R 33.02,0
32A_ATM = smd 1.5 x 0.4: 1 -4.25,2.8; 2 -4.25,2; 3 -4.25,1.2; 4 -4.25,0.4; 5 -4.25,-0.4; 6 -4.25,-1.2; 7 -4.25,-2; 8 -4.25,-2.8; 17 4.25,-2.8; 18 4.25,-2; 19 4.25,-1.2; 20 4.25,-0.4; 21 4.25,0.4; 22 4.25,1.2; 23 4.25,2; 24 4.25,2.8 | smd 0.4 x 1.5: 9 -2.8,-4.25; 10 -2,-4.25; 11 -1.2,-4.25; 12 -0.4,-4.25; 13 0.4,-4.25; 14 1.2,-4.25; 15 2,-4.25; 16 2.8,-4.25; 25 2.8,4.25; 26 2,4.25; 27 1.2,4.25; 28 0.4,4.25; 29 -0.4,4.25; 30 -1.2,4.25; 31 -2,4.25; 32 -2.8,4.25
SOT223 = smd 1.219 x 2.235: 1 -2.311,-3.099; 2 0,-3.099; 3 2.311,-3.099 | smd 3.6 x 2.2: 4.TAB 0,3.099
TXC7M2 = smd 1.2 x 1: 1 -1.2,-0.8; 2 1.2,-0.8; 3 1.2,0.8; 4 -1.2,0.8

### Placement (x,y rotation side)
$3_73_$  11.5,71.5 0 top
-  0,0 0 top
A1  83,91.5 0 top
A2  5,30 0 top
B1  21.5,10 0 top
B2  4.5,10 0 top
B3  32.5,68.5 270 top
B4  32.5,82 270 top
C1  53,23 90 top
C2  45.5,44 0 top
C3  45.5,42 0 top
C4  18,12 270 top
C5  86.5,72.5 270 top
C6  15.5,12 270 top
C7  59.1,61.3 180 top
C8  61.6,63.8 90 top
C9  53,64 270 top
C10  55,64 270 top
C11  43,67 0 top
C12  56.5,79.5 90 top
C13  43,79.5 0 top
C14  58.5,79.5 90 top
C15  43,73.5 0 top
C16  26,43.5 180 top
C17  26,41 180 top
C18  19,95 90 top
C19  22.5,95 90 top
C20  29.5,91.5 0 top
C21  28.5,82.5 0 top
C22  29.5,89.5 0 top
C23  28.5,80.5 0 top
C24  54.3,79.5 90 top
D1  13,92.5 180 top
D2  17,43.5 0 top
D3  17,36 0 top
D4  13,96 0 top
D5  17,41 0 top
D6  17,38.5 0 top
D7  13,89 0 top
J1  76,3.5 0 top
J2  96.5,21.5 270 top
J3  66.04,71.46 90 top
J4  58.36,91.46 0 top
J5  96.52,83.82 180 top
J6  35.5,91.46 0 top
J7  4.5,82 90 top
J8  5,39.5 0 top
LED1  50,17.5 0 top
LED2  69.54,59.46 180 top
LED3  26,36 0 top
R1  49,23 270 top
R2  47,23 270 top
R3  51,23 270 top
R4  26.5,18 180 top
R5  26.5,20 180 top
R6  88.5,72.5 270 top
R7  90.5,72.5 270 top
R8  26.5,24 0 top
R9  26.5,22 180 top
R10  43,65 180 top
R11  43,63 180 top
R12  69.54,61.46 0 top
R13  43,75.5 0 top
R14  43,77.5 180 top
R15  60.5,79.5 270 top
R16  26,38.5 180 top
U1  50,1.5 0 top
U2  19,32 0 top
U3  50,33 270 top
U4  96.5,73.65 270 top
U5  33.5,45 0 top
U6  54,72 90 top
U7  19,64.5 0 top
U8  22.5,89.5 90 top
U9  21.5,80.5 90 top
U$2  12.7,2.9 0 top
Y1  58.5,63.9 180 top

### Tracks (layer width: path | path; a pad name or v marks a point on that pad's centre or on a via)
3V3  (via drill 0.5 pad 0.9)
  Top 0.5: C22.1 U8.2 v22,89.5 U8.4.TAB 19.5,89.4 | v17,94.5 15.5,94.5 15.05,94.95 D4.A
  Bottom 0.5: v17,94.5 v22,89.5
5V0
  Top 0.5: D7.A 15.05,86.95 18.4,83.6 U9.4.TAB U9.2 C23.1
+3V3
  Top 0.5: D4.C 9.5,96 8.5,95 8.5,90.5 3,85 3,76.5 7,72.5 7,51.45 D2.C 7,43.5 5,41.5 J8.1 5,37 6,36 D3.C
+5V
  Top 0.5: D7.C 8.5,89 4,84.5 4,77 8,73 8,52 14.5,45.5 16,45.5 17,44.5 17,41.5 16.5,41 D5.C D6.C 13,38.5 12,39.5 J8.3
ADC6
  Top 0.3: U6.19 55.2,77.35 55.4,77.55 55.4,82.9 53.28,85.02 J6.8
  Bottom 0.5: J6.9 J6.8
ADC7
  Top 0.3: U6.22 52.8,77.4 51.1,79.1 51.1,81.01 50.74,81.37 J6.7
  Bottom 0.5: J6.10 J6.7
AREF
  Top 0.3: U6.20 54.4,77.4 54.3,77.5 C24.1
AT-USB-3V3
  Top 0.5: D2.A 19,43.55 19,45 10,54 10,63.5 11,64.5 U7.1.3V3
AT-USB-5V
  Top 0.5: D5.A 20.5,41 21,41.5 21,44.8 19,46.8 U7.6.5V
AT_DTR_CAP
  Top 0.3: U7.2.DTR 20.36,61.96 20.9,62.5 20.9,69.1 25.3,73.5 C15.1
AT_MISO  (via drill 0.5 pad 0.9)
  Top 0.3: U6.16 62.2,74.8 63,74 v62.98,73.98
  Bottom 0.3: v62.98,73.98 63,73.96 63,73 64.54,71.46 J3.1
AT_MOSI  (via drill 0.5 pad 0.9)
  Top 0.3: U6.15 59.5,74 60,73.5 v61,73.5
  Bottom 0.3: J3.4 66.97,75.61 61.62,75.61 61,75 v61,73.5
AT_RST  (via drill 0.5 pad 0.9)
  Top 0.3: R13.2 C15.2 43.95,72.4 44.51,71.84 v46.25,71.84 47.26,71.84 47.5,71.6 U6.29
  Bottom 0.3: J3.5 69.16,69.5 64.2,69.5 61.95,71.75 52.21,71.75 50.85,70.39 50.85,65.01 49.54,63.7 48.46,63.7 47.7,64.46 47.7,66.06 45.5,68.26 45.5,71.09 v46.25,71.84
AT_RST_CAP
  Top 0.3: R13.1 C13.1 R14.2
  Top 0.5: C13.1 41,79.5 39.5,79.5 B4.3.B B4.4.B
AT_RXD
  Top 0.3: U6.30 47.25,70.8 46.95,70.5 44.6,70.5 42.9,72.2 31.2,72.2 22,63 22,58 20.88,56.88 U7.4.RDO
AT_SCK
  Top 0.2: 56.8,69.2 57.7,68.3
  Top 0.3: J3.3 68.58,70.08 67.92,69.42 65.08,69.42 64.4,70.1 64.4,74.4 61.2,77.6 57.2,77.6 56.8,77.2 U6.17 56.8,69.2 | 57.7,68.3 60.72,68.3 63.45,65.57 65.73,65.57 68.6,62.7 R12.1
AT_TXD  (via drill 0.5 pad 0.9)
  Top 0.3: U6.31 47.55,70 47.35,69.8 44.4,69.8 42.55,71.65 31.43,71.65 23.5,63.72 v23.5,60.5
  Bottom 0.3: v23.5,60.5 22.42,59.42 U7.3.RXI
AVCC
  Top 0.3: U6.18 56,77.3 56.5,77.8 C12.1 C14.1 R15.2
B1-CAP
  Top 0.5: C4.1 19.55,14.5 B1.3.B B1.4.B 28,14.55 25.55,17 R4.2 R5.2
GND  (via drill 0.5 pad 0.9, 1.1)
  Top 0.3: U6.5 54.4,69.1 54,69.5 v53.6,69.5 53.2,69.5 52.8,69.1 U6.3 | v52.9,74.6 53.3,74.6 53.6,74.9 U6.21
  Top 0.5: C7.1 61.3,61.3 v61.5,61.5 61.6,61.6 C8.1
  other vias: 88.94,36.76 88.94,62.16 88.94,59.62 88.94,57.08 88.94,54.54 88.94,52 88.94,49.46 88.94,46.92 88.94,44.38 88.94,41.84 88.94,39.3 30.5,87.5 86.5,70 88.94,34.22 88.94,31.68 88.94,29.14 25,96 25,94 27,94 29,94 32.5,89.5 32.5,91.5 28,86.5 22,87.5 22,86 29.5,85 21,78.5 8,86.5 11,86.5 29.5,16.5 29.5,24.5 28.5,37 21.5,21 21.5,23 16.5,23 16.5,21 16,55.5 16,53.5 22,53.5 22,55.5 5.5,77.5 7,76 27,77.5 29.5,78.5 28.5,77.5 21,77 28.5,35 41,68.5 23,44 23,42 23,40 57.5,40.5 54.5,40.5 55,23.5 57,23.5 56,40.5 58.5,82.5 52,86 52,87.5 52,89 52.2,79.7 56.5,82.5 54.3,82.5 55.1,84.9 45.9,66.2 75.5,17.5 73.5,17.5 71.5,17.5 82.5,18.5 81,20 79.5,21.5 92.5,22.5 91,24 87.5,23.5 89,22 90.5,20.5 63,17 61,17 59,17 45,20 45,23 43,25 48,46 48,49 48,51.5 48,54 51,54 51,51.5 51,49 43,54 43,51.5 43,49 43,46 66.5,59.5 66.5,57.5 68,56.5 56,61 54,61 51.5,61 43,56.5 43,59 48,56.5 47.5,39 29,39.5 31.5,16.5 85,18.5 87.5,18.5 90,18.5 52.2,81.2 54.4,74.6 55.6,69.5 63.5,63 17,96 41,70 66.5,61.5 29.5,26.5 28,30.5 26.5,29 25,27.5 22,32.5 23.5,34 51,36.5 53,36.5 53,38 78,23 76.5,24.5 75,26 80,13 82,11 80,11 80,9 80,7 82,7 82,9 70,56.5 66,63 91,65.5 87.5,65.5 85,65.5 83,65.5 81,65.5 79,65.5 43.5,81.5 41.5,81.5 39.5,81.5 72,76.5 70,76.5 73.5,78.5 73.5,80.5 67.5,77 65,77 65.5,80.5 66.5,81.5 96.5,79 94.5,79 96.5,76 94.5,76 93.5,74.5 93,77.5 91.5,76 88,75.5 96,24.5 93.5,24.5 96,27 93.5,27 91,27 69.5,44 69.5,46 69.5,48 67.5,48 65.5,48 63.5,48 61.5,48 23,38 23,36 9.5,66.5 9.5,68.5 11,68.5 14,75.5 15.5,75.5 17.5,75.5 18.5,77 25.5,85 22,84.5 20,86 83.5,96.5 86,96.5 88.5,96.5 91,96.5 85.5,94.5 87.5,92.5 90,90 92.5,87.5 96.5,89.5 96.5,91.5 79.5,95 81.5,94 85.5,90 87.5,88 89.5,86 83.5,88 81,88 78.5,88 79.5,92 79.5,89.5 51.4,74.6
  pour Top (isolate 0.5): 2,2 98,2 98,98 2,98
  pour Bottom (isolate 0.5): 2,2 98,2 98,98 2,98
ICSP_CLK  (via drill 0.5 pad 0.9)
  Top 0.3: U3.18 58.17,36.17 61.92,39.92 U5.18.L U5.18.R 69.08,39.92 72.48,36.52 v72.48,28.52 | J1.5 86.16,10.84 74.5,22.5 v72.5,22.5
  Bottom 0.3: v72.5,22.5 72.5,28.5 v72.48,28.52
ICSP_DAT  (via drill 0.5 pad 0.9)
  Top 0.3: U3.19 57.45,37.45 62.46,42.46 U5.19.L U5.19.R 69.04,42.46 74,37.5 v74,27.5 | v74,20.5 75.5,20.5 83.62,12.38 J1.4
  Bottom 0.3: v74,20.5 v74,27.5
LED_POWER
  Top 0.5: R16.2 25.05,36.05 LED3.A
MCLR  (via drill 0.5 pad 0.9)
  Top 0.3: U5.4.L U5.4.R 39.12,37.38 41.59,34.91 U3.4 46.09,34.91 48,33 v48,30
  Top 0.5: R8.2 27.45,26.95 v31,30.5 | J1.1 76,12 79,15 79,16 76,19 63.5,19 56.5,26 54,26 53.5,26.5 v52.5,26.5
  Bottom 0.5: U5.4.L 31.88,37.38 31,36.5 v31,30.5 | v52.5,26.5 49,30 v48,30
MCLR_CAP
  Top 0.5: B2.3.B B2.4.B 13.95,14.5 C6.1 17,14.45 18,14.45 20.05,16.5 22,16.5 24,18.5 24,21.45 24.55,22 R9.2 R8.1
N$1  (via drill 1.1)  (1 unrouted)
  Top 0.5: v91.48,36.76 v96.56,36.76
  other vias: 94.02,36.76
N$2  (via drill 1.1)  (1 unrouted)
  Top 0.5: v91.48,39.3 v96.56,39.3
  other vias: 94.02,39.3
N$3  (via drill 1.1)  (1 unrouted)
  Top 0.5: v91.48,41.84 v96.56,41.84
  other vias: 94.02,41.84
N$4
  Top 0.5: LED1.2 48.4,18.1 48,18.5 48,19.5 49,20.5 R1.2
N$5
  Top 0.5: LED1.3 47.6,16.9 47,17.5 R2.2
N$6
  Top 0.5: LED1.1 51.6,18.1 52,18.5 52,19.5 51,20.5 R3.2
N$7  (via drill 1.1)  (1 unrouted)
  Top 0.5: v91.48,44.38 v96.56,44.38
  other vias: 94.02,44.38
N$8  (via drill 1.1)  (1 unrouted)
  Top 0.5: v91.48,46.92 v96.56,46.92
  other vias: 94.02,46.92
N$9  (via drill 1.1)  (1 unrouted)
  Top 0.5: v91.48,49.46 v96.56,49.46
  other vias: 94.02,49.46
N$10  (via drill 1.1)  (1 unrouted)
  Top 0.5: v91.48,52 v96.56,52
  other vias: 94.02,52
N$11  (via drill 1.1)  (1 unrouted)
  Top 0.5: v91.48,54.54 v96.56,54.54
  other vias: 94.02,54.54
N$12  (via drill 1.1)  (1 unrouted)
  Top 0.5: v91.48,57.08 v96.56,57.08
  other vias: 94.02,57.08
N$13  (via drill 1.1)  (1 unrouted)
  Top 0.5: v91.48,59.62 v96.56,59.62
  other vias: 94.02,59.62
N$14  (via drill 1.1)  (1 unrouted)
  Top 0.5: v91.48,62.16 v96.56,62.16
  other vias: 94.02,62.16
N$15
  Top 0.3: 60,63 60,61.5
N$16
  Top 0.3: 59.2,63.4 59,63.4 58,64.4 57.7,64.4
N$20  (via drill 1.1)  (1 unrouted)
  Top 0.5: v78.78,36.76 v83.86,36.76
  other vias: 81.32,36.76
N$21  (via drill 1.1)  (1 unrouted)
  Top 0.5: v78.78,39.3 v83.86,39.3
  other vias: 81.32,39.3
N$22  (via drill 1.1)  (1 unrouted)
  Top 0.5: v78.78,41.84 v83.86,41.84
  other vias: 81.32,41.84
N$23  (via drill 1.1)  (1 unrouted)
  Top 0.5: v78.78,44.38 v83.86,44.38
  other vias: 81.32,44.38
N$24  (via drill 1.1)  (1 unrouted)
  Top 0.5: v78.78,46.92 v83.86,46.92
  other vias: 81.32,46.92
N$25  (via drill 1.1)  (1 unrouted)
  Top 0.5: v78.78,49.46 v83.86,49.46
  other vias: 81.32,49.46
N$26  (via drill 1.1)  (1 unrouted)
  Top 0.5: v78.78,52 v83.86,52
  other vias: 81.32,52
N$27  (via drill 1.1)  (1 unrouted)
  Top 0.5: v78.78,54.54 v83.86,54.54
  other vias: 81.32,54.54
N$28  (via drill 1.1)  (1 unrouted)
  Top 0.5: v83.86,57.08 v78.78,57.08
  other vias: 81.32,57.08
N$29  (via drill 1.1)
  Top 0.3: v81.32,59.62 v83.86,59.62
  Top 0.5: v78.78,59.62 v83.86,59.62
N$30  (via drill 1.1)
  Top 0.5: v78.78,62.16 v81.32,62.16 v83.86,62.16
N$33  (via drill 1.1)
  Top 0.406: v83.86,71.08 v83.86,73.62 v83.86,76.16
  Bottom 0.5: v83.86,76.16 83.86,83.78 J5.6 J5.11
N$34  (via drill 1.1)
  Top 0.406: v81.32,71.08 v81.32,73.62 v81.32,76.16
  Bottom 0.5: v81.32,76.16 81.32,83.78 J5.7 J5.10
N$35  (via drill 1.1)
  Top 0.406: v78.78,71.08 v78.78,73.62 v78.78,76.16
  Bottom 0.5: v78.78,76.16 78.78,83.78 J5.8 J5.9
N$37
  Top 0.5: R12.2 70.49,59.51 LED2.A
N$39  (via drill 1.1)  (1 unrouted)
  Top 0.5: v78.78,29.14 v83.86,29.14
  other vias: 81.32,29.14
N$40  (via drill 1.1)  (1 unrouted)
  Top 0.5: v78.78,31.68 v83.86,31.68
  other vias: 81.32,31.68
N$41  (via drill 1.1)  (1 unrouted)
  Top 0.5: v78.78,34.22 v83.86,34.22
  other vias: 81.32,34.22
N$42  (via drill 1.1)  (1 unrouted)
  Top 0.5: v91.48,29.14 v96.56,29.14
  other vias: 94.02,29.14
N$43  (via drill 1.1)  (1 unrouted)
  Top 0.5: v91.48,31.68 v96.56,31.68
  other vias: 94.02,31.68
N$44  (via drill 1.1)  (1 unrouted)
  Top 0.5: v91.48,34.22 v96.56,34.22
  other vias: 94.02,34.22
PB0
  Top 0.3: U6.12 59.4,71.6 59.95,71.05 61.12,71.05 64.4,67.77 68.6,67.77 69.13,68.3 72.06,68.3 74.3,70.54 74.3,75.74 76.76,78.2 88.36,78.2 J5.14
  Bottom 0.5: J5.3 J5.14
PB1
  Top 0.3: U6.13 59.4,72.4 60.2,71.6 61.34,71.6 64.62,68.32 68.38,68.32 68.91,68.85 71.83,68.85 73.75,70.77 73.75,75.97 76.53,78.75 86.37,78.75 J5.13
  Bottom 0.5: J5.4 J5.13
PB2
  Top 0.3: U6.14 59.4,73.2 60.4,72.2 61.52,72.2 64.85,68.87 68.15,68.87 68.68,69.4 71.6,69.4 73.2,71 73.2,76.2 76.3,79.3 84.4,79.3 86.36,81.26 J5.12
  Bottom 0.5: J5.5 J5.12
PC0
  Top 0.3: U6.23 52,77.4 50.55,78.85 50.55,80.78 48.2,83.13 J6.6
  Bottom 0.5: J6.11 J6.6
PC1
  Top 0.3: U6.24 51.2,77.4 50,78.6 50,80.56 45.66,84.9 J6.5
  Bottom 0.5: J6.12 J6.5
PC2
  Top 0.3: U6.25 48.9,74.8 48.7,75 48.7,75.82 49.45,76.57 49.45,80.33 43.12,86.66 J6.4
  Bottom 0.5: J6.13 J6.4
PC3
  Top 0.3: U6.26 48.4,74 48.1,74.3 48.1,76 48.9,76.8 48.9,80.1 40.58,88.42 J6.3
  Bottom 0.5: J6.14 J6.3
PD2  (via drill 0.5 pad 0.9)
  Top 0.3: U6.32 48.4,69.2 v47.5,68.3 | J4.3 63.44,85.44 62.5,84.5 v62.5,81.5
  Bottom 0.3: v47.5,68.3 47.5,69.6 51.45,73.55 55.87,73.55 62.5,80.18 v62.5,81.5
  Bottom 0.5: J4.14 J4.3
PD3  (via drill 0.5 pad 0.9)
  Top 0.3: U6.1 51.2,66.8 50.5,66.1 49.9,66.1 v49,67 | J4.4 66,91.44 66,86 64,84 v64,82.5
  Bottom 0.3: v49,67 49,70.3 51.7,73 56.5,73 64,80.5 v64,82.5
  Bottom 0.5: J4.13 J4.4
PD4  (via drill 0.5 pad 0.9)
  Top 0.3: R10.1 v49,65 50.5,65 52,66.5 U6.2 | J4.5 68.52,87.02 65.3,83.8 65.3,81.96 64,80.66 v64,78.5
  Bottom 0.3: v49,65 50.2,66.2 50.2,70.62 51.98,72.4 57,72.4 63.1,78.5 v64,78.5
  Bottom 0.5: J4.12 J4.5
PD4-CAP
  Top 0.3: B3.4.B 39.5,62 40.5,63 R11.2 | C11.1 R10.2
  Top 0.5: R11.2 R10.2 | B3.4.B B3.3.B
PD5  (via drill 0.5 pad 0.9)
  Top 0.3: U6.9 60.6,69.2 63.68,66.12 69.29,66.12 69.82,66.65 72.74,66.65 75.09,69 v76.5,69
  Bottom 0.3: v76.5,69 75,70.5 75,73.22 74.45,73.77 74.45,76.23 74.86,76.64 74.86,85.64 71.06,89.44 J4.6
  Bottom 0.5: J4.11 J4.6
PD6  (via drill 0.5 pad 0.9)
  Top 0.3: U6.10 59.4,70 59.6,69.8 60.81,69.8 63.94,66.67 69.06,66.67 69.59,67.2 72.51,67.2 75.4,70.09 75.4,71.4 v76.5,72.5
  Bottom 0.3: v76.5,72.5 75,74 75,76 75.5,76.5 75.5,87.5 73.6,89.4 J4.7
  Bottom 0.5: J4.10 J4.7
PD7  (via drill 0.5 pad 0.9)
  Top 0.3: U6.11 59.4,70.8 59.7,70.5 60.89,70.5 64.17,67.22 68.83,67.22 69.36,67.75 72.28,67.75 74.85,70.32 74.85,74.5 75.35,75 v76.5,75
  Bottom 0.3: v76.5,75 76.5,89 76.14,89.36 J4.8
  Bottom 0.5: J4.9 J4.8
PIC-USB-3V3
  Top 0.5: D3.A 19.05,32.05 U2.1.3V3
PIC-USB-5V
  Top 0.5: D6.A 17.5,38.5 17,38 17,34.5 15,32.5 15,20.5 16.2,19.3 U2.6.5V
RA2
  Top 0.3: U3.17 58.91,34.91 61.38,37.38 U5.17.L U5.17.R
  Top 0.5: U3.17 52.41,34.91 50.5,33 50.5,27.98 51,27.48 R3.1
RA4
  Top 0.3: U3.3 42.33,36.17 38.58,39.92 U5.3.R U5.3.L
  Bottom 0.3: U1.1 35.64,14.86 31,19.5 31,27 29.5,28.5 29.5,34.16 29.8,34.46 29.8,37.8 31.92,39.92 U5.3.L
RA5  (via drill 0.5 pad 0.9)
  Top 0.3: U3.2 43.05,37.45 38.04,42.46 U5.2.R U5.2.L
  Top 0.5: R2.1 47,25 v46.5,25.5 | v49.5,26.5 49.5,35 47.05,37.45 U3.2
  Bottom 0.5: v46.5,25.5 47.5,26.5 v49.5,26.5
RB5
  Top 0.3: U3.12 57.45,28.55 61.32,24.68 U5.12.L U5.12.R 73.16,24.68 86.5,11.34 J2.5
RB7
  Top 0.3: U3.10 43.28,27.29 38.14,22.14 U5.10.R U5.10.L
  Top 0.5: U5.10.L 29.36,18 R4.1
RC0
  Top 0.3: U3.16 59.63,33.63 60.84,34.84 U5.16.L U5.16.R
  Bottom 0.3: U1.4 70,12.54 70,33 68.16,34.84 U5.16.R
RC1
  Top 0.3: U3.15 63.91,32.37 U5.15.L U5.15.R
  Bottom 0.3: U1.3 69,19.84 69,31.5 68.2,32.3 U5.15.R
RC2
  Top 0.3: U3.14 58.91,31.09 60.24,29.76 U5.14.L U5.14.R 69.24,29.76 82.58,16.42 J2.3
RC3  (via drill 0.5 pad 0.9)
  Top 0.3: U3.7 41.09,31.09 39.76,29.76 U5.7.R U5.7.L | v43.5,16 45,16 45.5,15.5 v77.5,15.5
  Bottom 0.3: U5.7.L 31.55,27.81 31.55,19.95 35.5,16 v43.5,16 | v77.5,15.5 93,15.5 94.62,13.88 J2.4
RC4
  Top 0.3: U3.6 36.1,32.37 U5.6.R U5.6.L
  Top 0.5: U2.3.RXI 21.42,26.92 26.8,32.3 U5.6.L
RC5  (via drill 0.5 pad 0.9)
  Top 0.3: U3.5 40.87,33.63 39.66,34.84 U5.5.R U5.5.L
  Top 0.5: U2.4.RDO 20.88,24.38 v22,25.5 | U5.5.L 31.84,34.84 30.5,33.5 26,33.5 v22,29.5
  Bottom 0.5: v22,29.5 v22,25.5
RC6
  Top 0.3: U3.8 41.83,29.82 39.22,27.22 U5.8.R U5.8.L
  Top 0.5: R1.1 49,25 47,27 47,29 46.17,29.82 U3.8
RC7
  Top 0.3: U3.9 42.55,28.55 38.68,24.68 U5.9.R U5.9.L
  Bottom 0.3: U5.9.R 38.32,24.68 45.34,17.66 U1.2
  Bottom 0.406: 45.34,10.16 U1.2
SCL  (via drill 0.5 pad 0.9)
  Top 0.3: $3_73_$.3.SCL 20.58,75.5 28.72,75.5 31.77,78.55 33.55,78.55 v34.5,79.5 | v47.5,79.5 46.2,78.2 46.2,76.96 46.95,76.21 46.95,73.55 48.1,72.4 U6.28 | U5.11.R U5.11.L 61.86,22.14 56.72,27.29 U3.11 53.72,27.29 52,29 v52,30 | v75.48,67.48 89.48,67.48 90.5,68.5 | v48,58.5 v48,61.5
  Top 0.5: U4.4 92.97,66.03 90.5,68.5 R7.2
  Bottom 0.3: v34.5,79.5 v47.5,79.5 48.9,78.1 48.9,76.8 48.3,76.2 45.87,76.2 43.5,73.83 43.5,63.16 45.16,61.5 v48,61.5 49.65,63.15 49.77,63.15 51.5,64.88 51.5,70.17 52.53,71.2 61.72,71.2 63.97,68.95 74.05,68.95 75.5,67.5 v75.48,67.48 | v52,30 50.5,31.5 50.5,32.72 49.24,33.98 49.24,57.26 v48,58.5
SDA  (via drill 0.5 pad 0.9)
  Top 0.3: $3_73_$.4.SDA 22.27,74.65 29.15,74.65 32,77.5 v34.5,77.5 | v47.5,77.5 47.5,74 48.3,73.2 U6.27 | U5.13.R U5.13.L 60.78,27.22 58.17,29.82 U3.13 54.17,29.82 53.5,30.5 53.5,31.5 53,32 v52,32 | v79.9,68.9 85.76,68.9 85.96,68.7 87.2,68.7 v88.5,70
  Top 0.5: U4.3 93.43,68.57 v92,70 | v88.5,70 R6.2
  Bottom 0.3: v34.5,77.5 35.5,78.5 46.5,78.5 v47.5,77.5 45.9,77.5 42.45,74.06 42.45,62.93 45.23,60.15 49.79,60.15 | v79.9,68.9 78.74,68.9 76.02,66.18 74.92,66.18 72.7,68.4 63.7,68.4 61.51,70.59 52.8,70.59 52.13,69.92 52.13,64.74 49.79,62.4 49.79,60.15 | v52,32 49.79,34.21 49.79,60.15
  Bottom 0.5: v92,70 v88.5,70
UNREG_IN
  Top 0.5: D1.A 11,92.5 13,90.5 13,86 13.79,85.21 J7.TIP
UNREG_IN_POLARITY_PROTECTED
  Top 0.5: C20.1 27.5,91.5 27.19,91.81 U8.3 23.69,91.81 22.5,93 C19.1 C18.1 17.45,92.5 D1.C 17.5,90.05 17.5,86.5 21.19,82.81 U9.3 26.19,82.81 26.5,82.5 C21.1
VDD  (via drill 0.5 pad 0.9, 1.1)
  Top 0.3: U3.1 43.28,38.72 43,39 43,40.45 C3.1 C2.1 | U5.1.L U5.1.R | U6.6 55.2,66.2 55,66 C10.1 | U6.4 53.6,66.6 53,66 C9.1 | J4.2 60.9,82 60.5,81.6 R15.1 61.55,80.45 62.5,79.5 62.5,77.54 J3.2
  Top 0.5: C16.1 27,43.55 27.05,43.5 29.5,43.5 31,45 U5.1.L | R16.1 C17.1 C16.1 | R5.1 R9.1 v29.5,22 | LED1.4 51.9,16.9 53,18 C1.1 54.45,22.05 v55,21.5 | $3_73_$.2.VDD 14.04,69.04 9,64 9,53 v15,47 | v8.5,34.5 11,34.5 13.95,31.55 13.95,19.99 16.29,17.65 20.65,17.65 v22,19 | C16.1 26.95,44.55 26,45.5 22.5,45.5 v21,47 | J1.2 78.54,11.46 v78,12 | J2.2 94.04,18.96 86.4,26.6 v86.4,29.14 v86.4,31.68 v86.4,34.22 v86.4,36.76 v86.4,39.3 v86.4,41.84 v86.4,44.38 v86.4,46.92 v86.4,49.46 v86.4,52 v86.4,54.54 v86.4,57.08 v86.4,59.62 v86.4,62.16 | U4.2 94.39,71.11 92.05,73.45 R7.1 R6.1 C5.1 86.5,76 87.55,77.05 88.63,77.05 90.58,79 91.7,79 J5.15 J5.2 81.3,96.5 61.8,96.5 60.9,95.6 | U5.1.R 41.5,45 v42.5,44 C2.1 44.55,60.45 43.95,61.05 R11.1 v45.5,63 50,63 51.95,64.95 C9.1 C10.1 | v45.65,73.64 45.65,76.01 44.76,76.9 44.55,76.9 R14.1 44.55,78.1 44.76,78.1 46,79.34 46,81.5 38.04,89.46 J6.2 J6.15 38.04,95.54 39,96.5 60,96.5 60.9,95.6 | 60.9,95.6 J4.15 J4.2
  Bottom 0.5: v8.5,34.5 7.54,35.46 J8.2 7.54,41.54 13,47 v15,47 v21,47 | v22,19 26.5,19 v29.5,22 | v86.4,62.16 86.4,63.4 87,64 93,64 94.5,65.5 94.5,70.5 95.11,71.11 U4.2 | v78,12 76,14 76,16 77,17 79,17 79.5,16.5 91.7,16.5 94.16,18.96 J2.2 | v42.5,44 42.5,27.5 48.5,21.5 v55,21.5 | v45.65,73.64 44.65,72.64 44.65,63.85 v45.5,63
XTAL1
  Top 0.25: C7.2 57.3,62.3 Y1.3
  Top 0.3: Y1.3 56.6,63.1 56.2,63.5 56.2,66.4 56,66.6 U6.7
XTAL2
  Top 0.25: C8.2 59.8,64.6 59.45,64.95
  Top 0.3: 59.6,64.8 59.7,64.9 59.7,65.4 58.6,66.5 57.1,66.5 56.8,66.8 U6.8 | 59.45,64.95 59.6,64.8 | 59.6,64.8 Y1.1 59.8,64.8

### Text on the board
tPlace: RESET | VDD | GND | PD4 | ATmega328P-AU | PIC16F1829 | 5V | 3V3 | VDD | GND | HELLO WORLD! | RESET | RB7
bPlace: REV A2
_tNames: D4 | D1 | C18 | C19 | C20 | D7 | C22 | U8 | C21 | C24 | C12 | C14 | R15 | C13 | J7 | C23 | R14 | U9 | R13 | C5 | R6 | R7 | C15 | J3 | U6 | C11 | R10 | C8 | R11 | R12 | C9 | C10 | Y1 | C7 | LED2 | D2 | C16 | C2 | J8 | C3 | D5 | C17 | U3 | D6 | R16 | D3 | LED3 | R8 | R9 | R2 | R1 | R3 | C1 | R5 | R4 | LED1 | C6 | C4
